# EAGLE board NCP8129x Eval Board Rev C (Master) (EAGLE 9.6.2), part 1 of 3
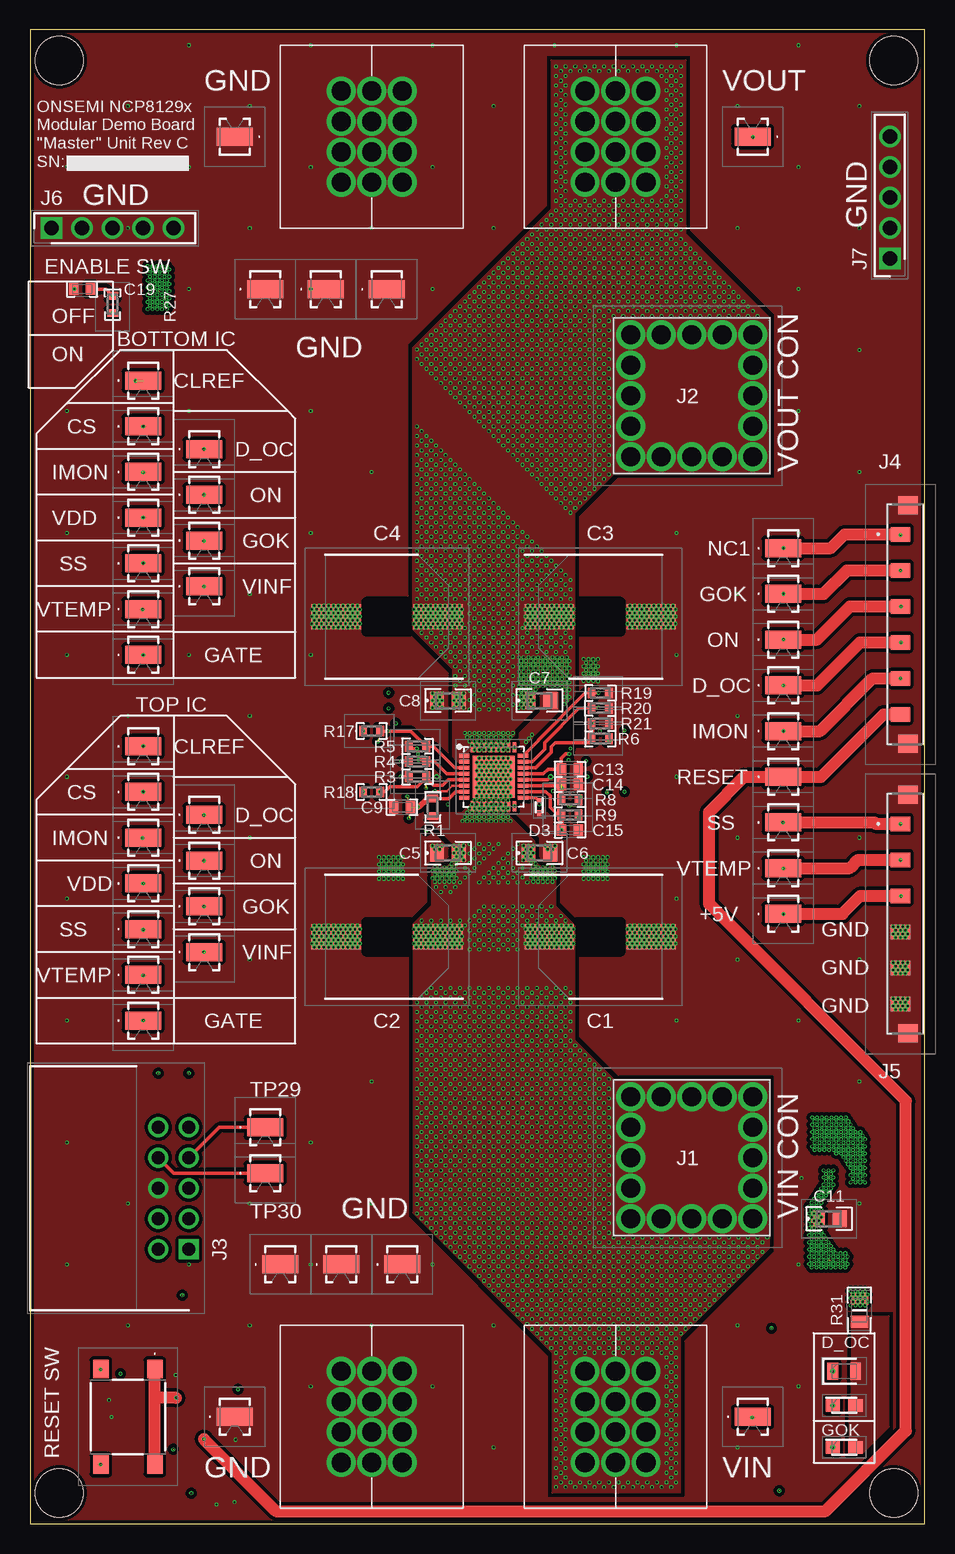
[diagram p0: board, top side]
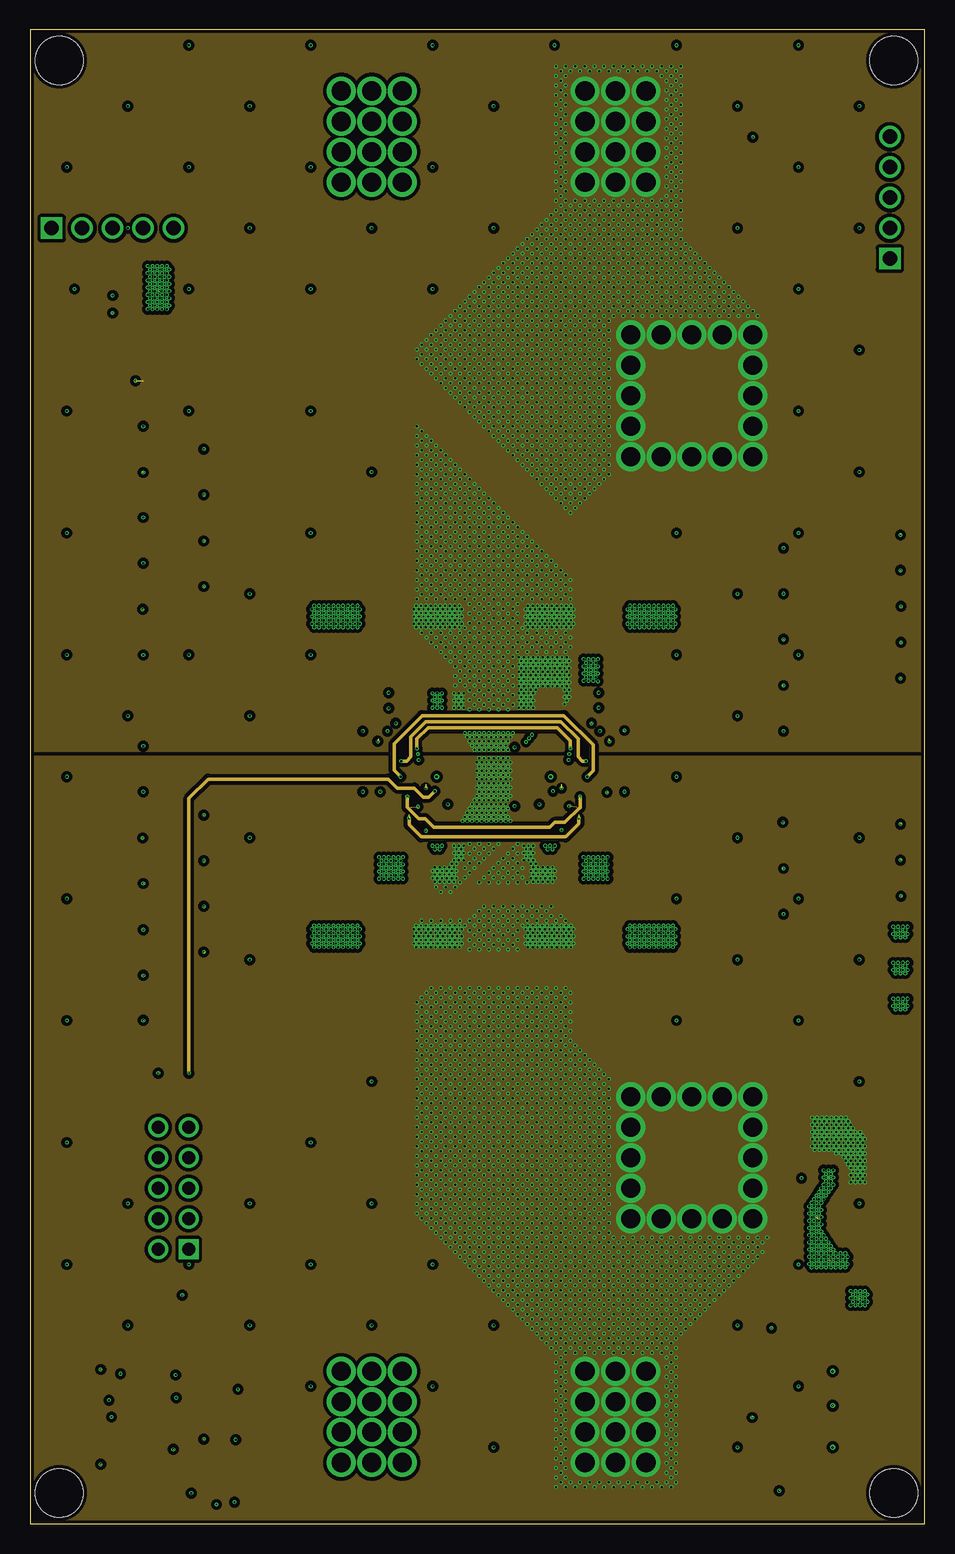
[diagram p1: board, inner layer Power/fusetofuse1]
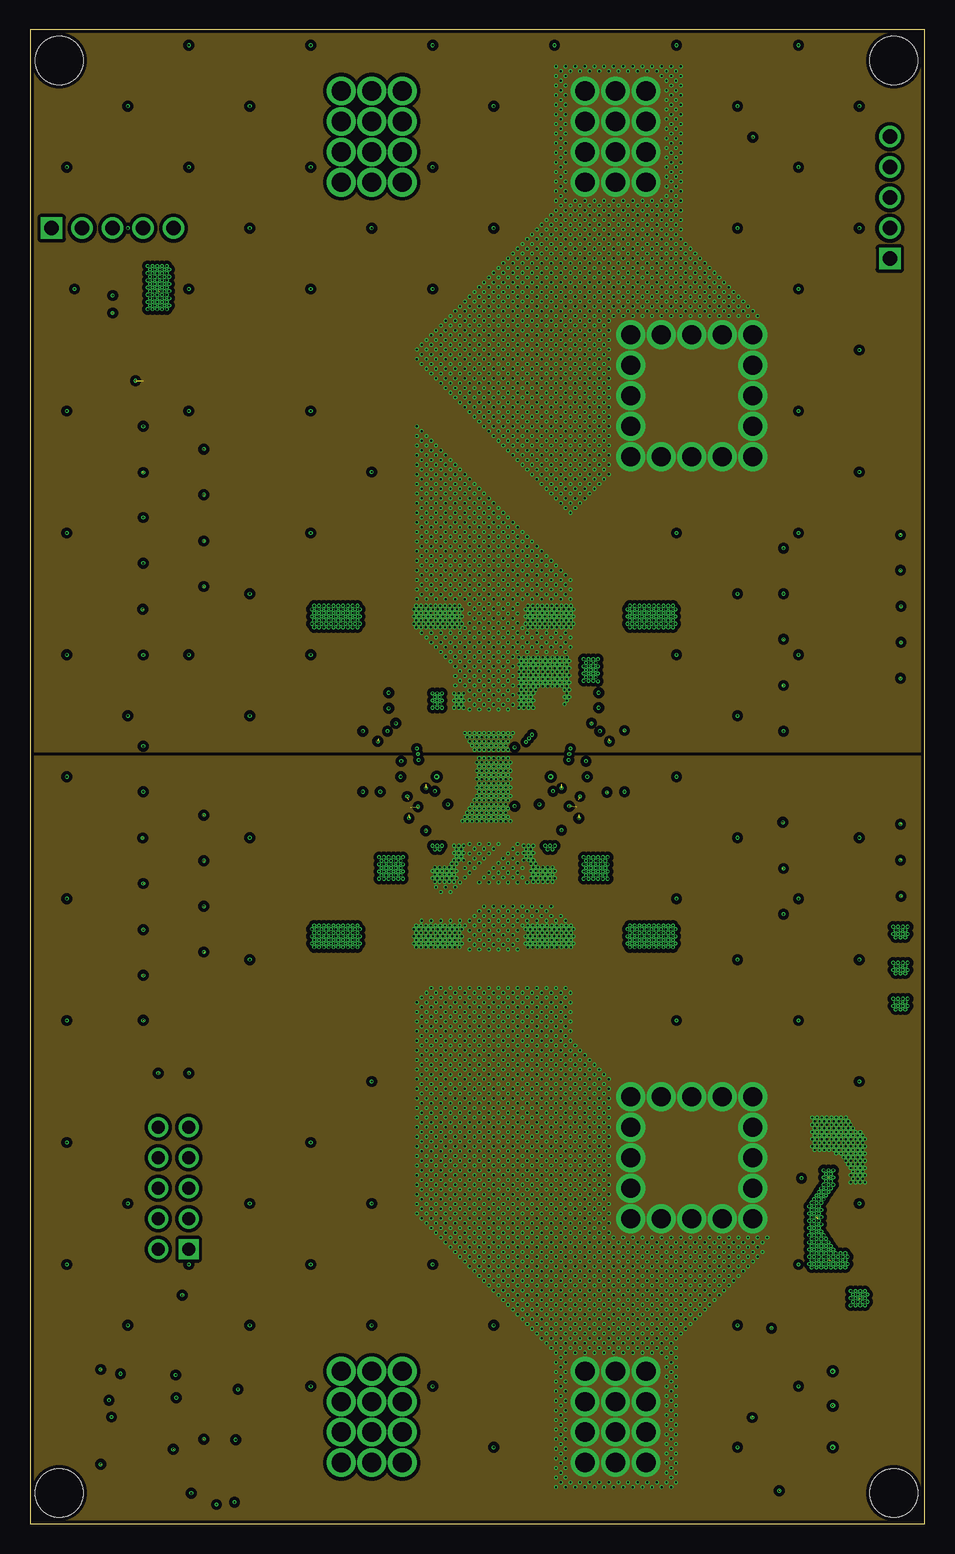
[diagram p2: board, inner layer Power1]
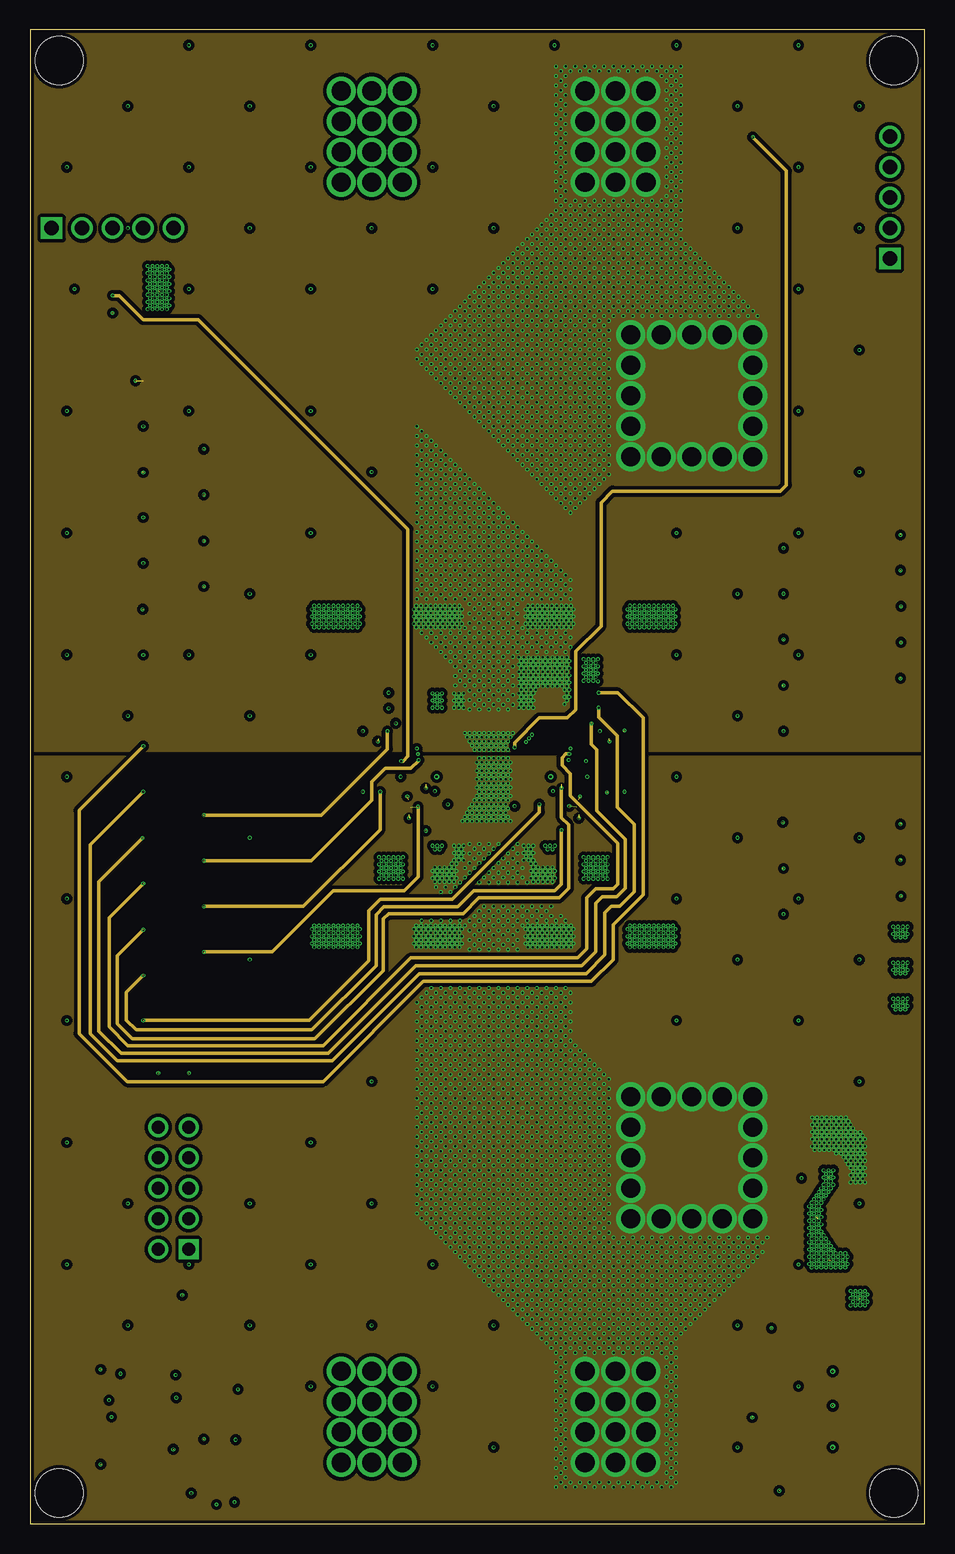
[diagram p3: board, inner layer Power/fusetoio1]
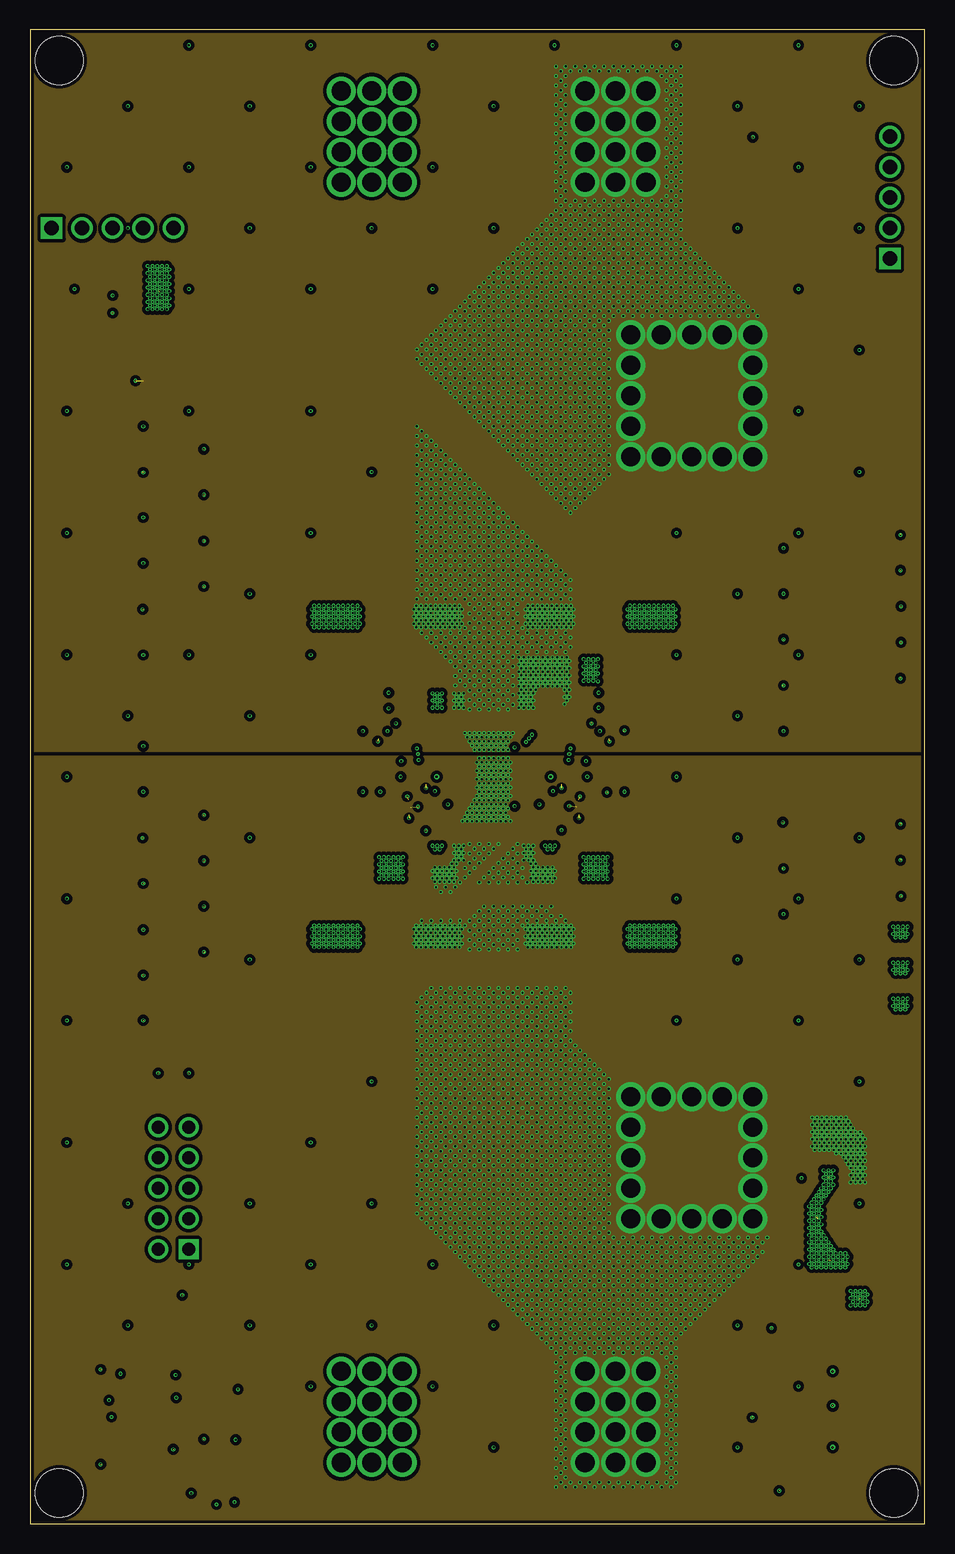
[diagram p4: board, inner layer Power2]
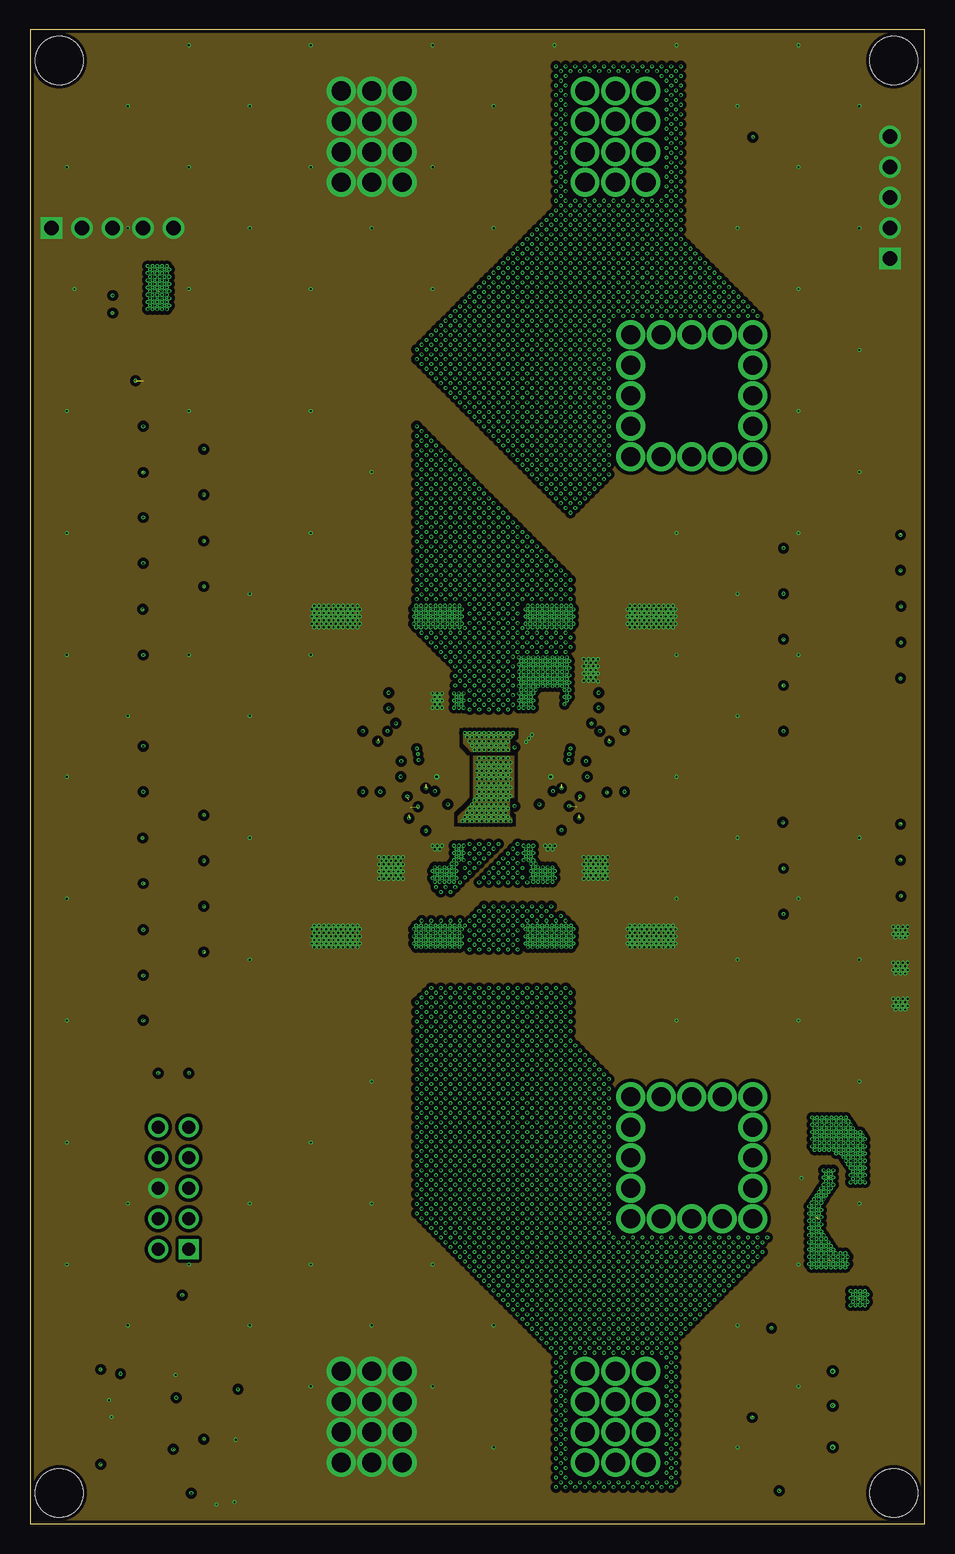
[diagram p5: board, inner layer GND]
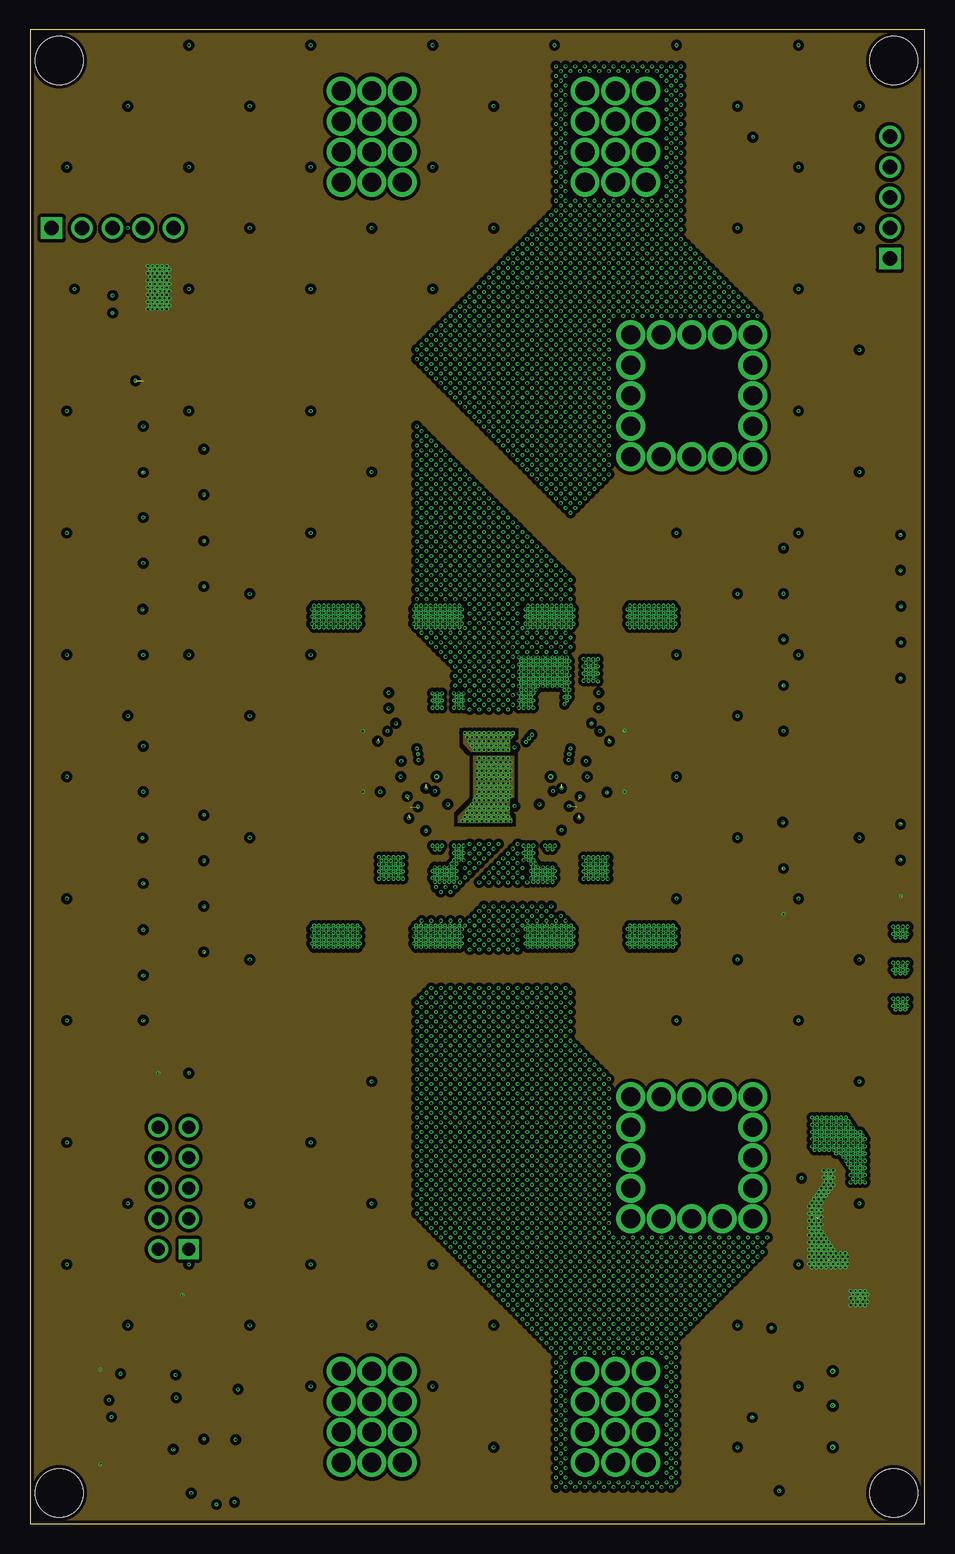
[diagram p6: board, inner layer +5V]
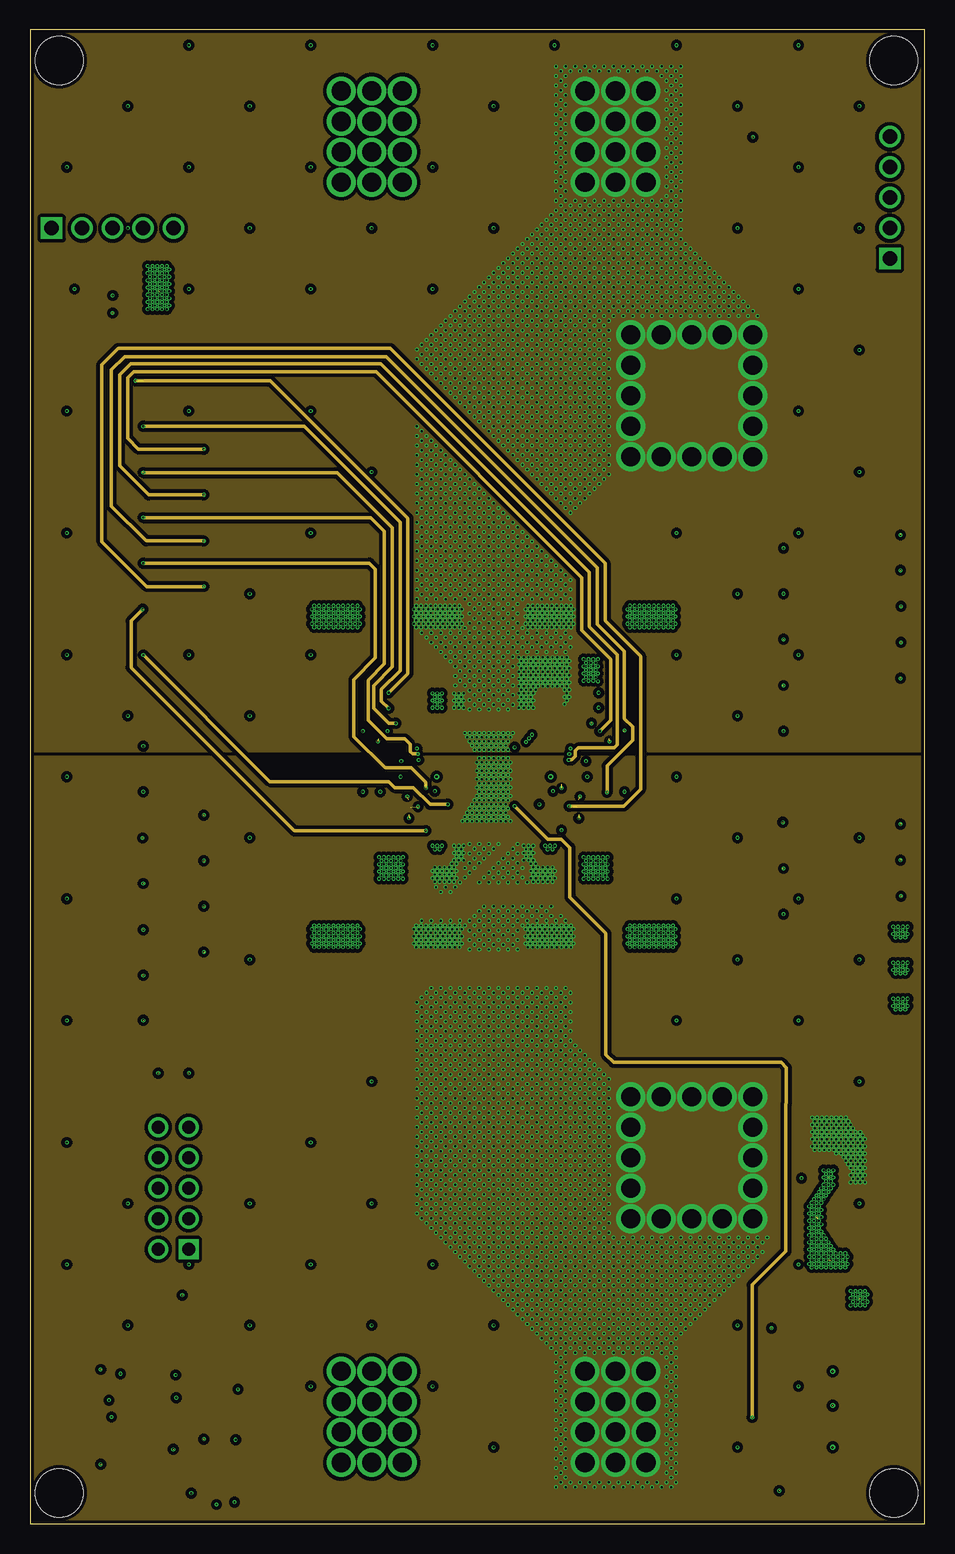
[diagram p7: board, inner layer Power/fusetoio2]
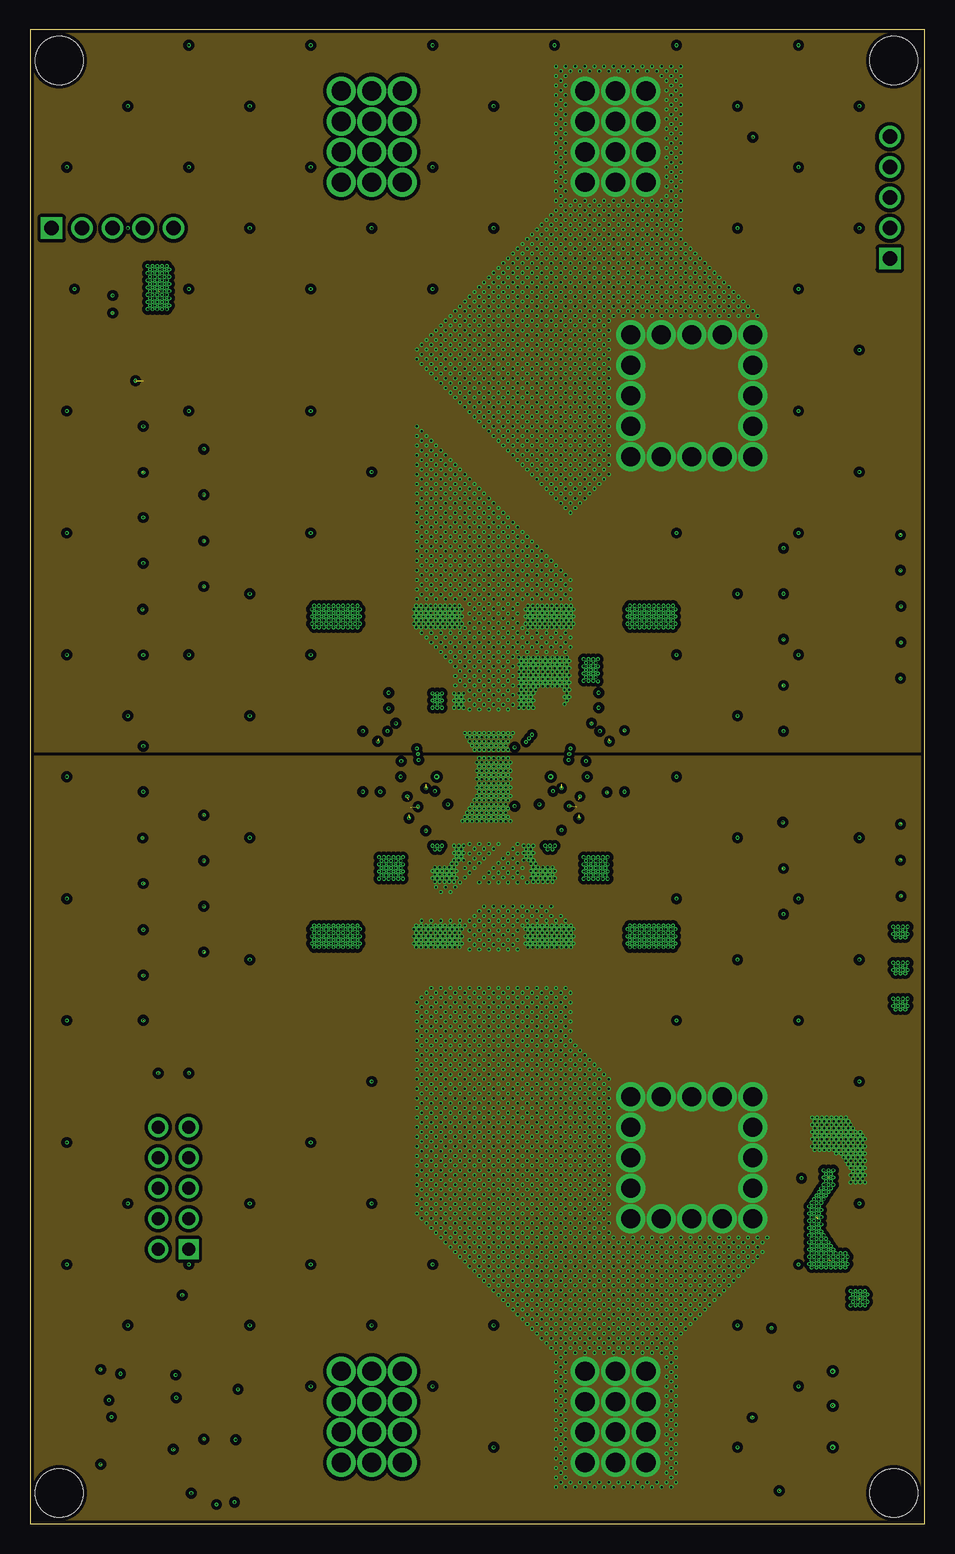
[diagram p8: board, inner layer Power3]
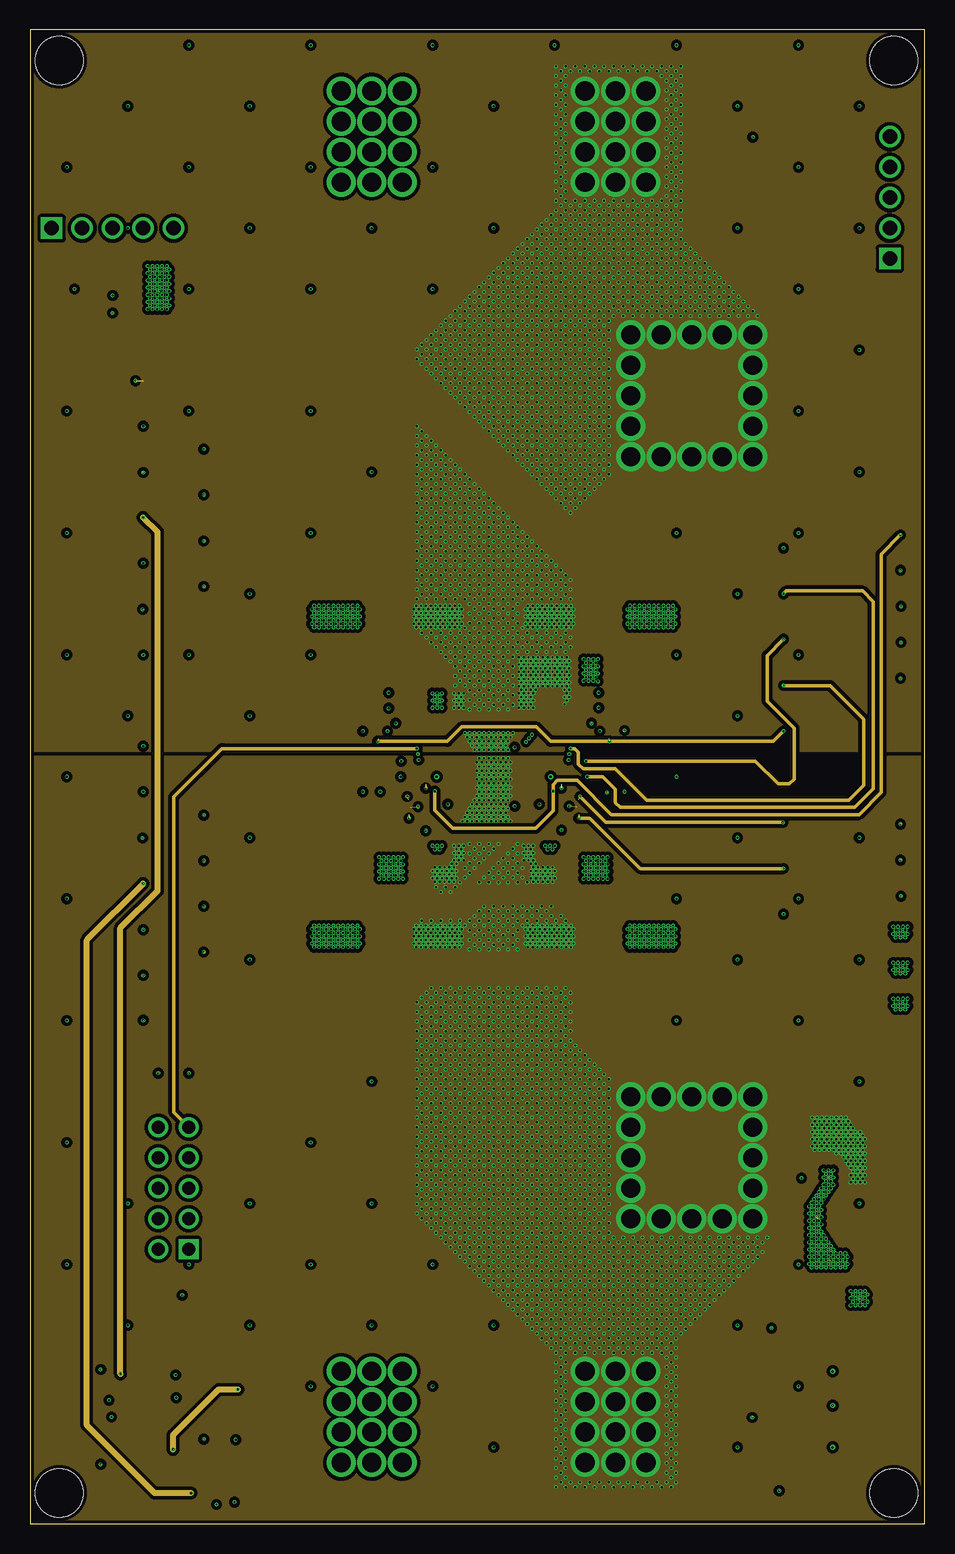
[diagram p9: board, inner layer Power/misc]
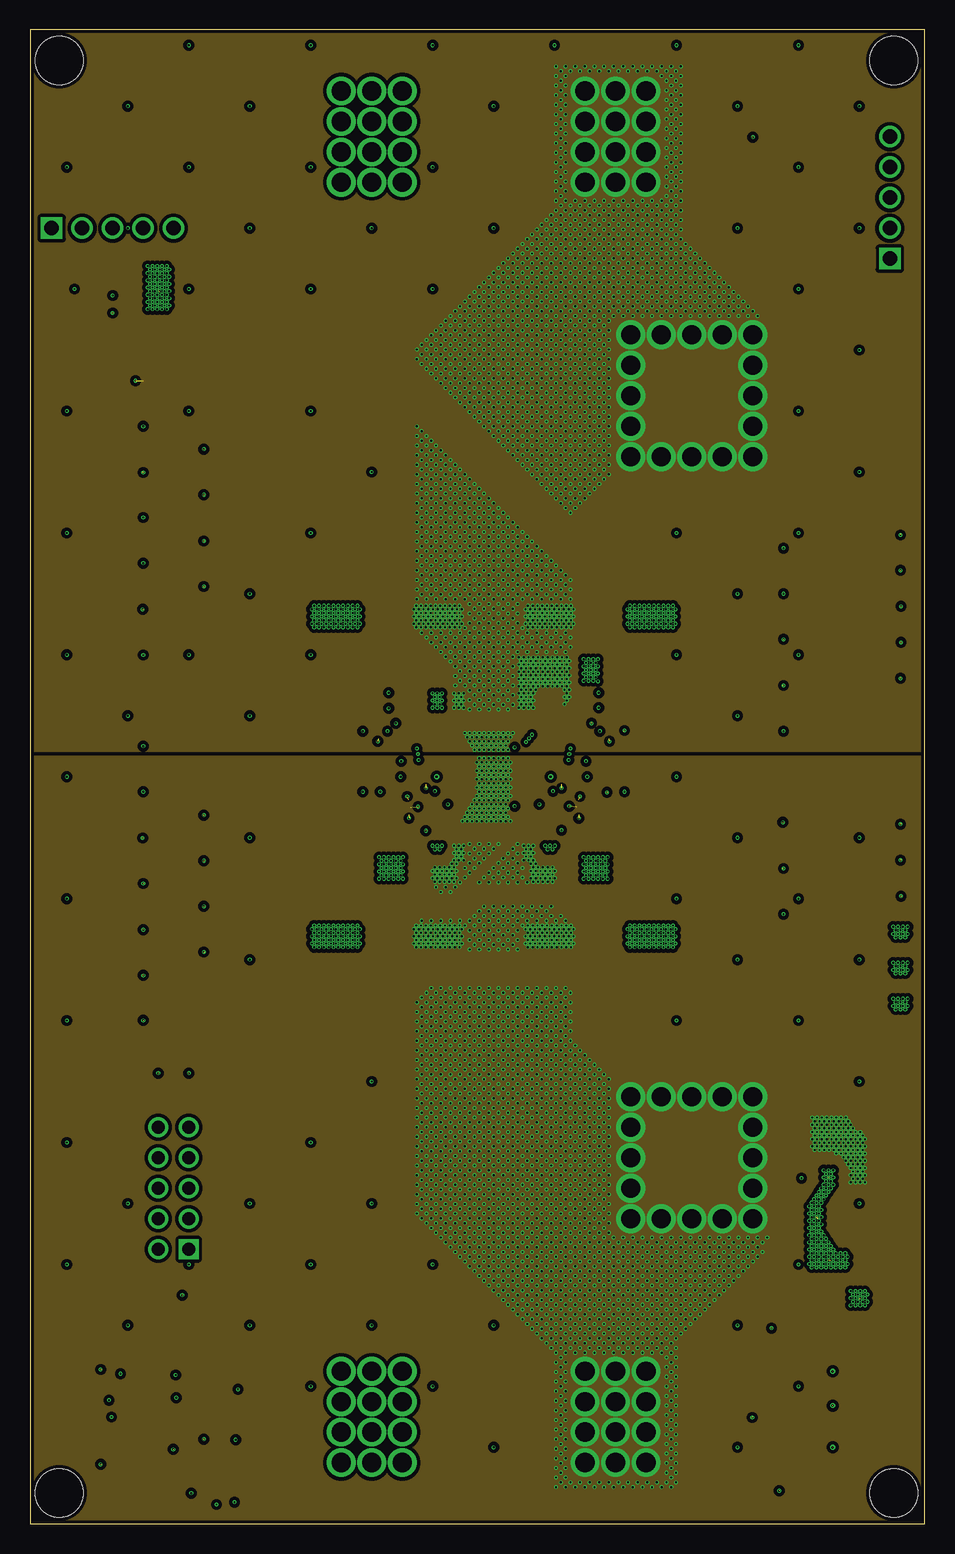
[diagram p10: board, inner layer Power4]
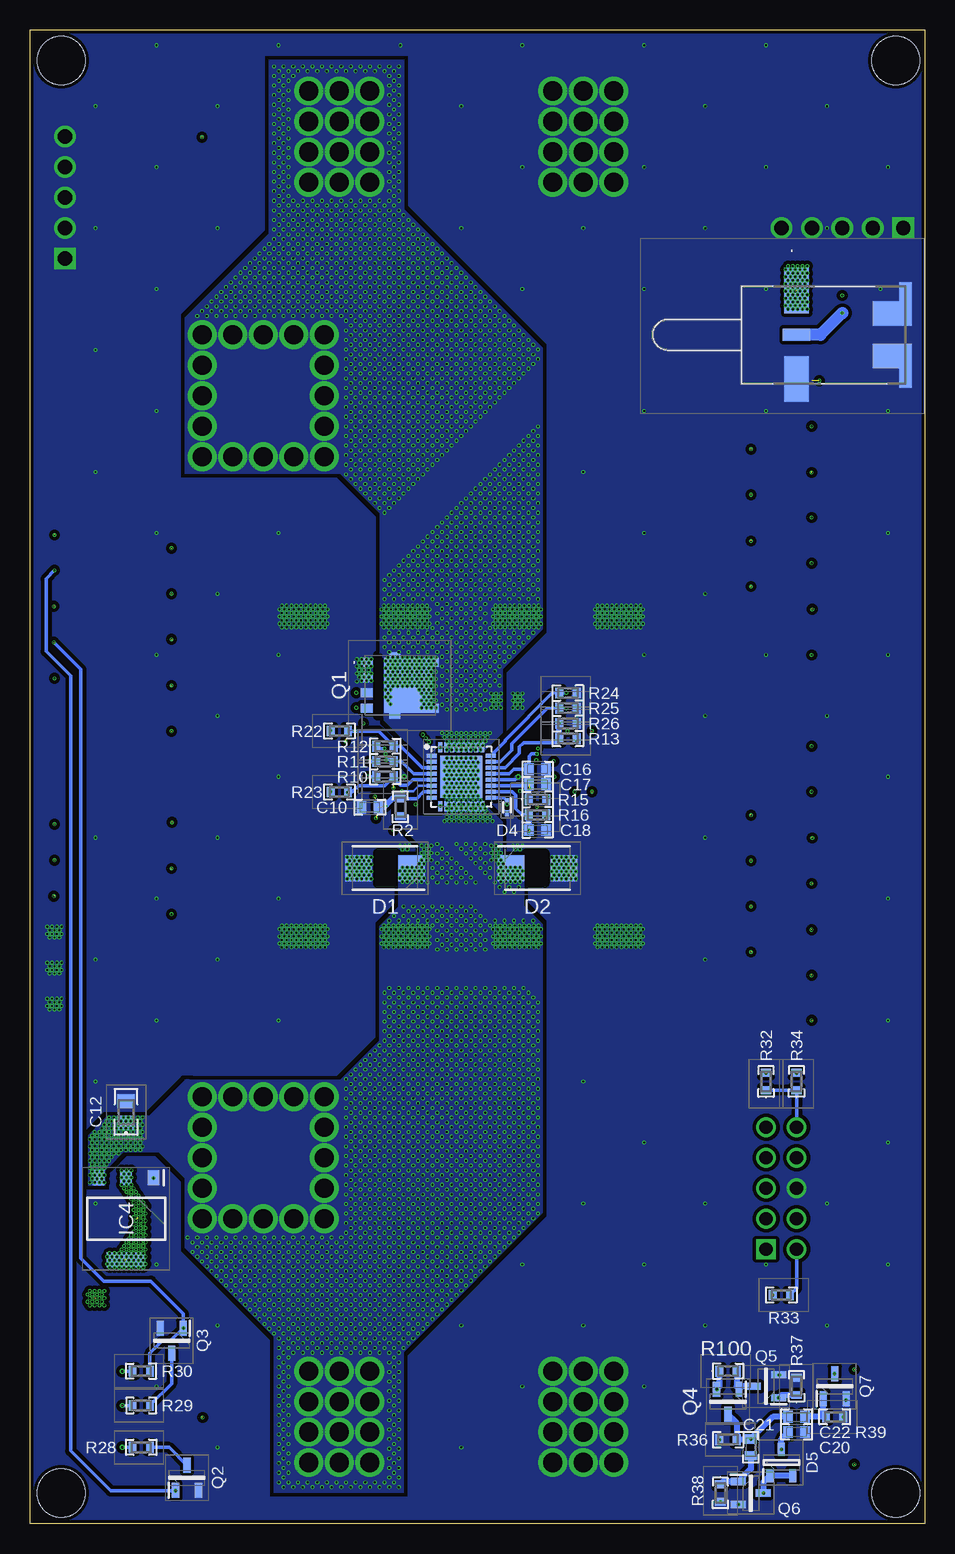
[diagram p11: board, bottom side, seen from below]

Size 74.57 x 124.46 mm. Coordinates in mm from the lower left corner, seen from the top.
Outline: 0,0 74.57,0 74.57,124.46 0,124.46 0,0
Copper layers (1+2*3+4*5+6*11+12*13+14*15+16): Top 0.035mm / dielectric 1.5mm / Power/fusetofuse1 0.035mm / dielectric 0.15mm / Power1 0.035mm / dielectric 0.2mm / Power/fusetoio1 0.035mm / dielectric 0.15mm / Power2 0.035mm / dielectric 0.2mm / GND 0.035mm / dielectric 0.15mm / +5V 0.035mm / dielectric 0.2mm / Power/fusetoio2 0.035mm / dielectric 0.15mm / Power3 0.035mm / dielectric 0.2mm / Power/misc 0.035mm / dielectric 0.15mm / Power4 0.035mm / dielectric 0.2mm / Bottom 0.035mm
Design rules "default *": minimum track width 1mil, minimum drill 0.35mm, track to track 6mil, track to pad 6mil, pad to pad 6mil, via to via 6mil, smd to smd 6mil, copper to edge 0.25mm, drill to drill 6mil, minimum pad ring 1mil, minimum via ring 1mil, stop-mask expansion 4mil, vias tented up to drill 0.3mm, thermal gap 10mil
Holes 4 mm at 2.44,121.92 71.97,121.92 2.44,2.54 71.97,2.54
tRestrict: area 28,47.6 to 31.6,50.2; area 45.6,47.6 to 49.3,50.2; area 28,74.3 to 31.6,76.8; area 45.6,74.3 to 49.3,76.8
bRestrict: area 31.6,53.3 to 33.2,55.9; area 44,53.3 to 45.6,55.9; area 45.3,67.3 to 45.6,72.4

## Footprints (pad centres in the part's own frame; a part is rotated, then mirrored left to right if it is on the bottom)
CAPAE1030X1050N = smd 4.1 x 2.05: 1 -4.25,0; 2 4.25,0
C0805 = smd 1.15 x 1.45: 1 -0.9,0; 2 0.9,0
CAPC1608X95N = smd 0.78 x 0.98: 1 -0.7,0; 2 0.7,0
DIOM5436X244N = smd 2.2 x 2.15: 1 -2.2,0; 2 2.2,0
SODFL1006X40N = smd 0.51 x 0.32: 1 -0.5,0; 2 0.5,0
SOT95P248X115-3N = smd 1.1 x 0.6: 1 -1.1,0.95; 2 -1.1,-0.95; 3 1.1,0
QFN50P500X500X140-33N = smd 0.85 x 0.3: 1 -2.45,1.75; 2 -2.45,1.25; 3 -2.45,0.75; 4 -2.45,0.25; 5 -2.45,-0.25; 6 -2.45,-0.75; 7 -2.45,-1.25; 8 -2.45,-1.75; 17 2.45,-1.75; 18 2.45,-1.25; 19 2.45,-0.75; 20 2.45,-0.25; 21 2.45,0.25; 22 2.45,0.75; 23 2.45,1.25; 24 2.45,1.75 | smd 0.3 x 0.85: 9 -1.75,-2.45; 10 -1.25,-2.45; 11 -0.75,-2.45; 12 -0.25,-2.45; 13 0.25,-2.45; 14 0.75,-2.45; 15 1.25,-2.45; 16 1.75,-2.45; 25 1.75,2.45; 26 1.25,2.45; 27 0.75,2.45; 28 0.25,2.45; 29 -0.25,2.45; 30 -0.75,2.45; 31 -1.25,2.45; 32 -1.75,2.45 | smd 3.5 x 3.5: 33 0,0
SOT230P700X180-4N = smd 1.25 x 0.95: 1 -3.4,2.3; 2 -3.4,0; 3 -3.4,-2.3 | smd 1.25 x 3.2: 4 3.4,0
7461059 = drill 1.6 pad 2.3: 1 0,0; 2 0,-2.54; 3 0,-5.08; 4 0,-7.62; 5 0,-10.16; 6 2.54,-10.16; 7 5.08,-10.16; 8 7.62,-10.16; 9 10.16,-10.16; 10 10.16,-7.62; 11 10.16,-5.08; 12 10.16,-2.54; 13 10.16,0; 14 7.62,0; 15 5.08,0; 16 2.54,0
SHDRRA10W64P254X254_2X5_2036X8 = drill 1.1 pad 1.65 square: 1 0,0 | drill 1.1 pad 1.65: 2 0,2.54; 3 2.54,0; 4 2.54,2.54; 5 5.08,0; 6 5.08,2.54; 7 7.62,0; 8 7.62,2.54; 9 10.16,0; 10 10.16,2.54
209159006101116 = smd 1.2 x 1.6: 1 -7.5,-0.38; 2 -4.5,-0.38; 3 -1.5,-0.38; 4 1.5,-0.38; 5 4.5,-0.38; 6 7.5,-0.38 | smd 1.5 x 1.6: MP1 -9.935,0.25; MP2 9.935,0.25
RHDR5W70P0X254_1X5_1310X250X86 = drill 1.2 pad 1.8 square: 1 0,0 | drill 1.2 pad 1.8: 2 2.54,0; 3 5.08,0; 4 7.62,0; 5 10.16,0
LEDM2012X80N = smd 1.2 x 1.05: 1 -0.95,0; 2 0.95,0
LEDC2012X80N = smd 0.9 x 1.4: 1 -0.95,0; 2 0.95,0
NTMFS006N12MCT1G = smd 0.75 x 1: 1 -1.905,-2.795; 2 -0.635,-2.795; 3 0.635,-2.795; 4 1.905,-2.795 | smd 4.56 x 0.425: 5 0,-1.118 | smd 5.55 x 0.905: 6 0,-0.453 | smd 4.56 x 2.725: 7 0,1.362 | smd 0.75 x 0.475: 8 1.905,2.962; 9 -1.905,2.962
SOT96P237X111-3N = smd 1.25 x 0.6: 1 -1.05,0.955; 2 -1.05,-0.955; 3 1.05,0
SOT95P237X101-3N = smd 1.25 x 0.6: 1 -1.05,0.95; 2 -1.05,-0.95; 3 1.05,0
ERJS03J155V = smd 0.65 x 0.9: 1 -0.725,0; 2 0.725,0
RESC2012X75N = smd 1 x 1.45: 1 -0.95,0; 2 0.95,0
ET01MD1SAPE = smd 3.81 x 2.03: 1 -3.685,0; 3 3.685,0 | smd 1.02 x 2.29: 2 0,0 | smd 3.63 x 1.02: MP1 -2.58,9.07; MP4 2.58,9.07 | smd 2.03 x 2.23: MP2 -1.78,7.445; MP3 1.78,7.445
430182043816 = smd 1.55 x 1.3: 1 -3.975,2.25; 2 -3.975,-2.25; 3 3.975,2.25; 4 3.975,-2.25
5191TR = smd 3 x 1.5: 1 0,0
7464000 = drill 1.6: P$1 0,2.54; P$2 0,0; P$3 0,-2.54; P$4 0,-5.08; P$5 2.54,-5.08; P$6 2.54,-2.54; P$7 2.54,0; P$8 2.54,2.54; P$9 5.08,2.54; P$10 5.08,0; P$11 5.08,-2.54; P$12 5.08,-5.08

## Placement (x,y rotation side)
C1  865230557006  [CAPAE1030X1050N]  47.52,48.89 0 top
C2  865230557006  [CAPAE1030X1050N]  29.74,48.89 180 top
C3  865230557006  [CAPAE1030X1050N]  47.52,75.56 0 top
C4  865230557006  [CAPAE1030X1050N]  29.74,75.56 180 top
C5  C0805X223K5RACTU  [C0805]  34.82,55.88 0 top
C6  C0805X223K5RACTU  [C0805]  42.44,55.88 0 top
C7  C0805X223K5RACTU  [C0805]  42.44,68.58 0 top
C8  C0805X223K5RACTU  [C0805]  34.82,68.58 0 top
C9  C0603C104K1RACAUTO  [CAPC1608X95N]  31.01,59.69 180 top
C10  C0603C104K1RACAUTO  [CAPC1608X95N]  46.25,59.69 180 bottom
C11  C0805X223K5RACTU  [C0805]  66.57,25.4 0 top
C12  C0805X223K5RACTU  [C0805]  66.57,34.29 90 bottom
C13  C0603C104K1RACAUTO  [CAPC1608X95N]  44.98,62.86 0 top
C14  C0603C104K1RACAUTO  [CAPC1608X95N]  44.98,61.59 0 top
C15  C0603C104K1RACAUTO  [CAPC1608X95N]  44.98,57.78 0 top
C16  C0603C104K1RACAUTO  [CAPC1608X95N]  32.28,62.86 0 bottom
C17  C0603C104K1RACAUTO  [CAPC1608X95N]  32.28,61.59 0 bottom
C18  C0603C104K1RACAUTO  [CAPC1608X95N]  32.28,57.78 0 bottom
C19  C0603C104K1RACAUTO  [CAPC1608X95N]  4.34,102.87 180 top
C20  C0603C104K1RACAUTO  [CAPC1608X95N]  10.69,7.62 0 bottom
C21  C0603C104K1RACAUTO  [CAPC1608X95N]  14.5,6.35 90 bottom
C22  C0603C104K1RACAUTO  [CAPC1608X95N]  10.69,8.89 180 bottom
D1  SMBJ13A  [DIOM5436X244N]  44.98,54.61 180 bottom
D2  SMBJ13A  [DIOM5436X244N]  32.28,54.61 0 bottom
D3  BAS16P2T5G  [SODFL1006X40N]  42.44,59.69 270 top
D4  BAS16P2T5G  [SODFL1006X40N]  34.82,59.69 270 bottom
D5  BAT54C-G3-08  [SOT95P248X115-3N]  11.96,5.08 90 bottom
IC1  NCP81295MNTXG  [QFN50P500X500X140-33N]  38.63,62.23 0 top
IC2  NCP81295MNTXG  [QFN50P500X500X140-33N]  38.63,62.23 0 bottom
IC4  LM1117MPX-18NOPB  [SOT230P700X180-4N]  66.57,25.4 270 bottom
J1  7461059  [7461059]  50.06,35.56 0 top
J2  7461059  [7461059]  50.06,99.06 0 top
J3  61201021721  [SHDRRA10W64P254X254_2X5_2036X8]  13.23,22.86 90 top
J4  209159006101116  [209159006101116]  72.92,74.93 270 top
J5  209159006101116  [209159006101116]  72.92,50.8 270 top
J6  M20-7820542  [RHDR5W70P0X254_1X5_1310X250X86]  1.8,107.95 0 top
J7  M20-7820542  [RHDR5W70P0X254_1X5_1310X250X86]  71.65,105.41 90 top
LED1  150080GS75000  [LEDM2012X80N]  67.84,6.35 0 top
LED2  150080GS75000  [LEDM2012X80N]  67.84,9.84 0 top
LED3  150080RS75000  [LEDC2012X80N]  67.84,12.7 0 top
Q1  NTMFS006N12MCT1G  [NTMFS006N12MCT1G]  43.71,69.85 270 bottom
Q2  2N7002LT1  [SOT96P237X111-3N]  61.49,3.81 90 bottom
Q3  2N7002LT1  [SOT96P237X111-3N]  62.76,15.24 270 bottom
Q4  NTR1P02LT1G  [SOT95P237X101-3N]  16.41,10.16 270 bottom
Q5  NTR3C21NZT1G  [SOT96P237X111-3N]  13.23,11.43 180 bottom
Q6  NTR3C21NZT1G  [SOT96P237X111-3N]  14.5,2.54 0 bottom
Q7  NTR3C21NZT1G  [SOT96P237X111-3N]  7.52,11.43 90 bottom
R1  ERJU03F56R0V  [ERJS03J155V]  33.55,59.69 270 top
R2  ERJU03F56R0V  [ERJS03J155V]  43.71,59.69 270 bottom
R3  ERJU03F56R0V  [ERJS03J155V]  32.28,62.23 0 top
R4  ERJU03F56R0V  [ERJS03J155V]  32.28,63.5 0 top
R5  ERJU03F56R0V  [ERJS03J155V]  32.28,64.77 0 top
R6  ERJU03F56R0V  [ERJS03J155V]  47.52,65.41 0 top
R8  ERJU03F56R0V  [ERJS03J155V]  44.98,60.32 0 top
R9  ERJU03F56R0V  [ERJS03J155V]  44.98,59.05 0 top
R10  ERJU03F56R0V  [ERJS03J155V]  44.98,62.23 0 bottom
R11  ERJU03F56R0V  [ERJS03J155V]  44.98,63.5 0 bottom
R12  ERJU03F56R0V  [ERJS03J155V]  44.98,64.77 0 bottom
R13  ERJU03F56R0V  [ERJS03J155V]  29.74,65.41 0 bottom
R15  ERJU03F56R0V  [ERJS03J155V]  32.28,60.32 0 bottom
R16  ERJU03F56R0V  [ERJS03J155V]  32.28,59.05 0 bottom
R17  ERJU03F56R0V  [ERJS03J155V]  28.47,66.04 0 top
R18  ERJU03F56R0V  [ERJS03J155V]  28.47,60.96 0 top
R19  ERJU03F56R0V  [ERJS03J155V]  47.52,69.22 0 top
R20  ERJU03F56R0V  [ERJS03J155V]  47.52,67.94 0 top
R21  ERJU03F56R0V  [ERJS03J155V]  47.52,66.67 0 top
R22  ERJU03F56R0V  [ERJS03J155V]  48.79,66.04 0 bottom
R23  ERJU03F56R0V  [ERJS03J155V]  48.79,60.96 0 bottom
R24  ERJU03F56R0V  [ERJS03J155V]  29.74,69.22 0 bottom
R25  ERJU03F56R0V  [ERJS03J155V]  29.74,67.94 0 bottom
R26  ERJU03F56R0V  [ERJS03J155V]  29.74,66.67 0 bottom
R27  ERJU03F56R0V  [ERJS03J155V]  6.88,101.6 90 top
R28  ERJU03F56R0V  [ERJS03J155V]  65.3,6.35 0 bottom
R29  ERJU03F56R0V  [ERJS03J155V]  65.3,9.84 0 bottom
R30  ERJU03F56R0V  [ERJS03J155V]  65.3,12.7 0 bottom
R31  ERJP6WF1303V  [RESC2012X75N]  69.11,17.78 270 top
R32  ERJU03F56R0V  [ERJS03J155V]  13.23,36.83 90 bottom
R33  ERJU03F56R0V  [ERJS03J155V]  11.96,19.05 180 bottom
R34  ERJU03F56R0V  [ERJS03J155V]  10.69,36.83 90 bottom
R36  ERJU03F56R0V  [ERJS03J155V]  16.41,6.98 180 bottom
R37  ERJU03F56R0V  [ERJS03J155V]  10.69,11.43 90 bottom
R38  ERJU03F56R0V  [ERJS03J155V]  17.04,2.54 270 bottom
R39  ERJU03F56R0V  [ERJS03J155V]  7.52,8.89 0 bottom
R100  ERJU03F56R0V  [ERJS03J155V]  16.41,12.7 0 bottom
S1  ET01MD1SAPE  [ET01MD1SAPE]  10.69,99.06 270 bottom
S2  430182043816  [430182043816]  8.15,8.89 270 top
TP1  5191TR  [5191TR]  19.58,33.02 0 top
TP2  5191TR  [5191TR]  19.58,29.21 0 top
TP3  5191TR  [5191TR]  17.04,8.89 0 top
TP4  5191TR  [5191TR]  60.22,8.89 0 top
TP5  5191TR  [5191TR]  17.04,115.57 180 top
TP6  5191TR  [5191TR]  60.22,115.57 180 top
TP7  5191TR  [5191TR]  62.76,81.28 0 top
TP8  5191TR  [5191TR]  62.76,77.47 0 top
TP9  5191TR  [5191TR]  62.76,73.66 0 top
TP10  5191TR  [5191TR]  62.76,69.85 0 top
TP11  5191TR  [5191TR]  62.76,66.04 0 top
TP12  5191TR  [5191TR]  62.76,62.23 0 top
TP13  5191TR  [5191TR]  62.76,58.42 0 top
TP14  5191TR  [5191TR]  62.76,54.61 0 top
TP15  5191TR  [5191TR]  14.5,59.05 0 top
TP16  5191TR  [5191TR]  14.5,55.24 0 top
TP17  5191TR  [5191TR]  14.5,51.43 0 top
TP18  5191TR  [5191TR]  14.5,47.62 0 top
TP19  5191TR  [5191TR]  9.42,41.91 0 top
TP20  5191TR  [5191TR]  9.42,45.72 0 top
TP21  5191TR  [5191TR]  9.42,49.53 0 top
TP22  5191TR  [5191TR]  9.42,53.34 0 top
TP23  5191TR  [5191TR]  9.42,57.15 0 top
TP24  5191TR  [5191TR]  9.42,60.96 0 top
TP25  5191TR  [5191TR]  9.42,64.77 0 top
TP26  5191TR  [5191TR]  14.5,89.53 0 top
TP27  5191TR  [5191TR]  14.5,85.72 0 top
TP28  5191TR  [5191TR]  14.5,81.91 0 top
TP29  5191TR  [5191TR]  14.5,78.1 0 top
TP30  5191TR  [5191TR]  9.42,72.39 0 top
TP31  5191TR  [5191TR]  9.42,76.2 0 top
TP32  5191TR  [5191TR]  9.42,80.01 0 top
TP33  5191TR  [5191TR]  9.42,83.82 0 top
TP34  5191TR  [5191TR]  9.42,87.63 0 top
TP35  5191TR  [5191TR]  9.42,91.44 0 top
TP36  5191TR  [5191TR]  9.42,95.25 0 top
TP37  5191TR  [5191TR]  62.76,50.8 0 top
TP38  5191TR  [5191TR]  19.58,102.87 0 top
TP39  5191TR  [5191TR]  24.66,102.87 0 top
TP40  5191TR  [5191TR]  29.74,102.87 0 top
TP41  5191TR  [5191TR]  20.85,21.59 0 top
TP42  5191TR  [5191TR]  25.93,21.59 0 top
TP43  5191TR  [5191TR]  31.01,21.59 0 top
U$1  7464000  [7464000]  25.93,10.16 0 top
U$2  7464000  [7464000]  46.25,10.16 0 top
U$3  7464000  [7464000]  25.93,116.84 0 top
U$4  7464000  [7464000]  46.25,116.84 0 top

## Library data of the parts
C1-C4 = SamacSys_Parts; DESCRIPTION: Wurth Elektronik 100uF 35 V dc Aluminium Electrolytic Capacitor, WCAP-AS5H Series 5000h 10.5 (Dia.) x 9.85mm; HEIGHT: 10.5mm; MANUFACTURER_NAME: Wurth Elektronik; MANUFACTURER_PART_NUMBER: 865230557006; MOUSER_PART_NUMBER: 710-865230557006; MOUSER_PRICE-STOCK: https://www.mouser.co.uk/ProductDetail/Wurth-Elektronik/865230557006?qs=0KOYDY2FL28VdE9DUGoPjQ%3D%3D
C5-C8 C11 C12 = SamacSys_Parts; ARROW_PART_NUMBER: C0805X223K5RACTU; ARROW_PRICE-STOCK: https://www.arrow.com/en/products/c0805x223k5ractu/kemet-corporation?region=nac; DESCRIPTION: SMD Comm X7R Flex, Ceramic, 0.022 uF, 10%, 50 VDC, 125 VDC, 125?C, -55?C, X7R, SMD, MLCC, FT-CAP, Temperature Stable, 2.5 % , 45.4545 GOhms, 13 mg, 0805, 2mm, 1.25mm, 0.78mm, 0.75mm, 0.5mm, 4000, 78 Weeks, 80; HEIGHT: 1.1mm; MANUFACTURER_NAME: KEMET; MANUFACTURER_PART_NUMBER: C0805X223K5RACTU; MOUSER_PART_NUMBER: 80-C0805X223K5R; MOUSER_PRICE-STOCK: https://www.mouser.co.uk/ProductDetail/KEMET/C0805X223K5RACTU?qs=p6yRp5s%252B%2FXRyuzEkovIpgw%3D%3D
C9 C10 C13-C22 = SamacSys_Parts; DESCRIPTION: SMD Auto X7R, Ceramic, 0.1 uF, 10%, 100 VDC, X7R, SMD, MLCC, Temperature Stable, Automotive Grade, 0603; HEIGHT: 0.95mm; MANUFACTURER_NAME: KEMET; MANUFACTURER_PART_NUMBER: C0603C104K1RACAUTO; MOUSER_PART_NUMBER: 80-C0603C104K1RAUTO; MOUSER_PRICE-STOCK: https://www.mouser.co.uk/ProductDetail/KEMET/C0603C104K1RACAUTO?qs=3Rah4i%252BhyCGTQ5uPNXtfZA%3D%3D
D1 D2 = SamacSys_Parts; DESCRIPTION: Diode TVS Single Uni-Dir 13V 600W 2-Pin SMB T/R; HEIGHT: 2.44mm; MANUFACTURER_NAME: LITTELFUSE; MANUFACTURER_PART_NUMBER: SMBJ13A; MOUSER_PART_NUMBER: 576-SMBJ13A; MOUSER_PRICE-STOCK: https://www.mouser.co.uk/ProductDetail/Littelfuse/SMBJ13A?qs=HR2RnyOI4E7jYyaNBU0w0w%3D%3D
D3 D4 = SamacSys_Parts; DESCRIPTION: Diodes - General Purpose, Power, Switching SWITCHING DIODE SOD923; HEIGHT: 0.4mm; MANUFACTURER_NAME: onsemi; MANUFACTURER_PART_NUMBER: BAS16P2T5G; MOUSER_PART_NUMBER: 863-BAS16P2T5G; MOUSER_PRICE-STOCK: https://www.mouser.co.uk/ProductDetail/onsemi/BAS16P2T5G?qs=xGcJQ%252BnsJwsOIzUKPy5pxg%3D%3D
D5 = SamacSys_Parts; DESCRIPTION: Vishay BAT54C-G3-08, Dual SMT Schottky Small Signal Diode, Common Cathode, 30V 200mA, 5ns, 3-Pin SOT-23; HEIGHT: 1.15mm; MANUFACTURER_NAME: Vishay; MANUFACTURER_PART_NUMBER: BAT54C-G3-08; MOUSER_PART_NUMBER: 78-BAT54C-G3-08; MOUSER_PRICE-STOCK: https://www.mouser.co.uk/ProductDetail/Vishay-Semiconductors/BAT54C-G3-08?qs=KP8Io%2FXyE5QQ%2FZAl3kVl1Q%3D%3D
IC1 IC2 = SamacSys_Parts; ARROW_PART_NUMBER: NCP81295MNTXG; ARROW_PRICE-STOCK: https://www.arrow.com/en/products/ncp81295mntxg/on-semiconductor; DESCRIPTION: HOT SWAP SMART FUSE; HEIGHT: 1.4mm; MANUFACTURER_NAME: onsemi; MANUFACTURER_PART_NUMBER: NCP81295MNTXG; MOUSER_PART_NUMBER: 863-NCP81295MNTXG; MOUSER_PRICE-STOCK: https://www.mouser.co.uk/ProductDetail/onsemi/NCP81295MNTXG?qs=W0yvOO0ixfEM9uhw2julAQ%3D%3D
IC4 = SamacSys_Parts; DESCRIPTION: Available in 1.8 V, 2.5 V, 3.3 V, 5 V, and Adjustable Versions; Space-saving SOT-223 package; Current limiting and thermal protection; Output current: 800 mA; Line regulation: 0.2% (maximum); Load regulation: 0.4% (maximum); HEIGHT: 1.8mm; MANUFACTURER_NAME: onsemi; MANUFACTURER_PART_NUMBER: LM1117MPX-18NOPB; MOUSER_PART_NUMBER: 863-LM1117MPX-18NOPB; MOUSER_PRICE-STOCK: https://www.mouser.co.uk/ProductDetail/onsemi/LM1117MPX-18NOPB?qs=DPoM0jnrROWLfPqSDvF0mA%3D%3D
J1 J2 = SamacSys_Parts; DESCRIPTION: Wurth Elektronik, Brass Screw Terminal, 240A; HEIGHT: 13.5mm; MANUFACTURER_NAME: Wurth Elektronik; MANUFACTURER_PART_NUMBER: 7461059; MOUSER_PART_NUMBER: 710-7461059; MOUSER_PRICE-STOCK: https://www.mouser.co.uk/ProductDetail/Wurth-Elektronik/7461059?qs=wr8lucFkNMXpCcsX18jYrg%3D%3D
J3 = SamacSys_Parts; DESCRIPTION: 10way 2.54mm male box Header right angle Wurth Elektronik WR-BHD Series, 2.54mm Pitch 10 Way 2 Row Shrouded Right Angle PCB Header, Surface Mount; HEIGHT: 9.1mm; MANUFACTURER_NAME: Wurth Elektronik; MANUFACTURER_PART_NUMBER: 61201021721; MOUSER_PART_NUMBER: 710-61201021721; MOUSER_PRICE-STOCK: https://www.mouser.co.uk/ProductDetail/Wurth-Elektronik/61201021721?qs=ZtY9WdtwX5567gkupD2iFg%3D%3D
J4 J5 = SamacSys_Parts; DESCRIPTION: Board to Board & Mezzanine Connectors Horizontal Sockt6Way 3mm Pitch 5A 125VAC; HEIGHT: 3mm; MANUFACTURER_NAME: Kyocera AVX; MANUFACTURER_PART_NUMBER: 209159006101116; MOUSER_PART_NUMBER: 581-209159006101116; MOUSER_PRICE-STOCK: https://www.mouser.co.uk/ProductDetail/KYOCERA-AVX/209159006101116?qs=b4vKS93X7SwcdpXWffJnjQ%3D%3D
J6 J7 = SamacSys_Parts; DESCRIPTION: Headers & Wire Housings 5 PIN SIL VERTICAL SOCKET GOLD+TIN; HEIGHT: 8.65mm; MANUFACTURER_NAME: Harwin; MANUFACTURER_PART_NUMBER: M20-7820542; MOUSER_PART_NUMBER: 855-M20-7820542; MOUSER_PRICE-STOCK: https://www.mouser.co.uk/ProductDetail/Harwin/M20-7820542?qs=vF78I%252BjhbY9JoekBTXVWnQ%3D%3D
LED1 LED2 = SamacSys_Parts; DESCRIPTION: 150080GS75000, Wurth Elektronik WL-SMCW 520 nm Green LED, 2012 (0805) Clear SMD package; HEIGHT: 0.8mm; MANUFACTURER_NAME: Wurth Elektronik; MANUFACTURER_PART_NUMBER: 150080GS75000; MOUSER_PART_NUMBER: 710-150080GS75000; MOUSER_PRICE-STOCK: https://www.mouser.co.uk/ProductDetail/Wurth-Elektronik/150080GS75000?qs=2kOmHSv6VfQRoTEZVk1mGA%3D%3D
LED3 = SamacSys_Parts; DESCRIPTION: LED,Wurth Elektronik,150080RS75000 Wurth Elektronik 150080RS75000, WL-SMCW Series Red LED, 625 nm 2012 (0805) Clear, Rectangle Lens SMD package; HEIGHT: 0.8mm; MANUFACTURER_NAME: Wurth Elektronik; MANUFACTURER_PART_NUMBER: 150080RS75000; MOUSER_PART_NUMBER: 710-150080RS75000; MOUSER_PRICE-STOCK: https://www.mouser.co.uk/ProductDetail/Wurth-Elektronik/150080RS75000?qs=LlUlMxKIyB2jdCo7bnfgew%3D%3D
Q1 = SamacSys_Parts; DESCRIPTION: ON Semiconductor NTMFS006N12MCT1G; HEIGHT: 1.1mm; MANUFACTURER_NAME: onsemi; MANUFACTURER_PART_NUMBER: NTMFS006N12MCT1G; MOUSER_PART_NUMBER: 863-NTMFS006N12MCT1G; MOUSER_PRICE-STOCK: https://www.mouser.co.uk/ProductDetail/onsemi/NTMFS006N12MCT1G?qs=HBWAp0VN4Ri6NIfu80r37A%3D%3D
Q2 Q3 = SamacSys_Parts; DESCRIPTION: MOSFET N-CH 60V 115MA SOT23-3; HEIGHT: 1.11mm; MANUFACTURER_NAME: onsemi; MANUFACTURER_PART_NUMBER: 2N7002LT1; MOUSER_PART_NUMBER: 863-2N7002LT1; MOUSER_PRICE-STOCK: https://www.mouser.co.uk/ProductDetail/onsemi/2N7002LT1?qs=vLkC5FC1VN%2FcwI%252Bf34Z4TQ%3D%3D
Q4 = SamacSys_Parts; DESCRIPTION: Small Signal MOSFET -20V -1.3A 220 mOhm Single P-Channel SOT-23 Logic Level; HEIGHT: 1.01mm; MANUFACTURER_NAME: onsemi; MANUFACTURER_PART_NUMBER: NTR1P02LT1G; MOUSER_PART_NUMBER: 863-NTR1P02LT1G; MOUSER_PRICE-STOCK: https://www.mouser.co.uk/ProductDetail/onsemi/NTR1P02LT1G?qs=ZXBb0xZ9WeCGH3oHt9wcQg%3D%3D
Q5-Q7 = SamacSys_Parts; DESCRIPTION: ON SEMICONDUCTOR - NTR3C21NZT1G - MOSFET, N-CH, 20V, 3.6A, SOT-23; HEIGHT: 1.11mm; MANUFACTURER_NAME: onsemi; MANUFACTURER_PART_NUMBER: NTR3C21NZT1G; MOUSER_PART_NUMBER: 863-NTR3C21NZT1G; MOUSER_PRICE-STOCK: https://www.mouser.co.uk/ProductDetail/onsemi/NTR3C21NZT1G?qs=tCMd4XlZ%2FiDqlfJKftdpPA%3D%3D
R1-R6 R8-R13 R15-R30 R32-R34 R36-R39 R100 = SamacSys_Parts; DESCRIPTION: Panasonic ERJU03 Series Thick Film Resistor 0603 Case 56 0.1W +/-100ppm/C; HEIGHT: 0.55mm; MANUFACTURER_NAME: Panasonic; MANUFACTURER_PART_NUMBER: ERJU03F56R0V
R31 = SamacSys_Parts; ARROW_PART_NUMBER: ERJP6WF1303V; ARROW_PRICE-STOCK: https://www.arrow.com/en/products/erj-p6wf1303v/panasonic; DESCRIPTION: Panasonic ERJP6W Series Thick Film Surface Mount Fixed Resistor 0805 Case 130k +/-1% 0.5W +/-200ppm/C; HEIGHT: 0.75mm; MANUFACTURER_NAME: Panasonic; MANUFACTURER_PART_NUMBER: ERJP6WF1303V
S1 = SamacSys_Parts; DESCRIPTION: Toggle Switches ON None ON SPDT 20VAC 20VDC 0.4W; HEIGHT: 5.72mm; MANUFACTURER_NAME: C & K COMPONENTS; MANUFACTURER_PART_NUMBER: ET01MD1SAPE; MOUSER_PART_NUMBER: 611-ET01MD1SAPE; MOUSER_PRICE-STOCK: https://www.mouser.co.uk/ProductDetail/CK/ET01MD1SAPE?qs=pYvtfcBFDEzTOYrckHtWUQ%3D%3D
S2 = SamacSys_Parts; DESCRIPTION: Black Tactile Switch, Single Pole Single Throw (SPST) 50 mA @ 12 V dc 0.9mm Surface Mount; HEIGHT: 4.45mm; MANUFACTURER_NAME: Wurth Elektronik; MANUFACTURER_PART_NUMBER: 430182043816; MOUSER_PART_NUMBER: 710-430182043816; MOUSER_PRICE-STOCK: https://www.mouser.co.uk/ProductDetail/Wurth-Elektronik/430182043816?qs=wr8lucFkNMVm%252BwK7rSM84A%3D%3D
TP1-TP43 = SamacSys_Parts; DESCRIPTION: Circuit Board Hardware - PCB TEST POINT (BLACK) ON TAPE AND REEL; HEIGHT: 2.63mm; MANUFACTURER_NAME: Keystone Electronics; MANUFACTURER_PART_NUMBER: 5191TR; MOUSER_PART_NUMBER: 534-5191TR; MOUSER_PRICE-STOCK: https://www.mouser.co.uk/ProductDetail/Keystone-Electronics/5191TR?qs=vLWxofP3U2z5ZV%2FXGVtphA%3D%3D
U$1-U$4 = SamacSys_Parts

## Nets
+5V: C11.1 IC4.2 IC4.4 J5.3 R17.1 R18.1 R22.1 R23.1 R31.1 R33.2 R34.2 S1.1 S2.2 S2.4 TP37.1
+5V_LED: LED1.2 LED2.2 LED3.2 R31.2
CLREF1: IC1.24 R19.1 TP25.1
CLREF2: IC2.24 R24.1 TP36.1
CS1: IC1.23 R20.1 TP24.1
CS2: IC2.23 R25.1 TP35.1
D_OC: J3.9 J4.4 Q3.1 R5.1 R12.1 R30.2 TP10.1
D_OC1: IC1.3 R5.2 R17.2 TP15.1
D_OC2: IC2.3 R12.2 R22.2 TP26.1
GATE1: D3.1 IC1.17 TP19.1
GATE2: D4.1 IC2.17 TP30.1
GND: C1.2 C2.2 C3.2 C4.2 C5.1 C6.2 C7.2 C8.1 C9.2 C10.2 C11.2 C12.2 C13.2 C14.2 C15.2 C16.2 C17.2 C18.2 C19.2 C20.2 D1.2 D2.2 D3.2 D4.2 IC1.20 IC2.20 IC4.1 J3.6 J4.MP1 J4.MP2 J5.4 J5.5 J5.6 J5.MP1 J5.MP2 J6.1 J6.2 J6.3 J6.4 J6.5 J7.1 J7.2 J7.3 J7.4 J7.5 Q1.1 Q1.2 Q1.3 Q2.2 Q3.2 Q5.2 Q6.2 Q7.2 R19.2 R20.2 R21.2 R24.2 R25.2 R26.2 R36.2 R37.2 R38.2 R39.2 S1.3 S1.MP1 S1.MP2 S1.MP3 S1.MP4 TP3.1 TP5.1 TP38.1 TP39.1 TP40.1 TP41.1 TP42.1 TP43.1 U$1.P$1 U$1.P$2 U$1.P$3 U$1.P$4 U$1.P$5 U$1.P$6 U$1.P$7 U$1.P$8 U$1.P$9 U$1.P$10 U$1.P$11 U$1.P$12 U$3.P$1 U$3.P$2 U$3.P$3 U$3.P$4 U$3.P$5 U$3.P$6 U$3.P$7 U$3.P$8 U$3.P$9 U$3.P$10 U$3.P$11 U$3.P$12
GOK: J4.2 Q2.1 R3.1 R10.1 TP8.1
GOK1: IC1.5 R3.2 R18.2 TP17.1
GOK2: IC2.5 R10.2 R23.2 TP28.1
IMON: J4.5 R6.2 R13.2 TP11.1
IMON1: IC1.22 R6.1 R21.1 TP23.1
IMON2: IC2.22 R13.1 R26.1 TP34.1
MASTER_RESET: Q5.1 R37.1 S2.1 S2.3
N$1: LED1.1 R28.1
N$2: Q2.3 R28.2
N$3: Q3.3 R29.2
N$4: LED2.1 R29.1
N$5: LED3.1 R30.1
N$6: J3.10 R32.1 R34.1
N$7: J3.2 R33.1
N$8: C20.1 D5.3 Q4.2 R100.1
N$9: Q4.1 Q5.3 R100.2
N$11: C21.1 Q6.1 R38.1
N$12: C22.1 Q7.1 R39.1
ON: C19.1 J4.3 R4.1 R11.1 R27.2 TP9.1
ON1: IC1.4 R4.2 TP16.1
ON2: IC2.4 R11.2 TP27.1
ON_PRE_RES: R27.1 S1.2
SDA: IC1.6 IC2.6 J4.1 R32.2 TP7.1
SLAVE_RESET: C21.2 C22.2 J4.6 Q4.3 R36.1 TP12.1
SS: J5.1 R8.2 R15.2 TP13.1
SS1: C14.1 IC1.19 R8.1 TP21.1
SS2: C17.1 IC2.19 R15.1 TP32.1
TP29: J3.7 TP1.1
TP30: J3.8 TP2.1
VDD1: C13.1 D5.1 D5.2 IC1.21 Q6.3 TP22.1
VDD2: C16.1 IC2.21 Q7.3 TP33.1
VIN: C1.1 C2.1 C5.2 C6.1 C12.1 D1.1 D2.1 IC1.9 IC1.10 IC1.11 IC1.12 IC1.13 IC1.14 IC1.15 IC1.33 IC2.10 IC2.11 IC2.12 IC2.13 IC2.14 IC2.15 IC2.16 IC2.33 IC4.3 J1.1 J1.2 J1.3 J1.4 J1.5 J1.6 J1.7 J1.8 J1.9 J1.10 J1.11 J1.12 J1.13 J1.14 J1.15 J1.16 R1.2 R2.2 U$2.P$1 U$2.P$2 U$2.P$3 U$2.P$4 U$2.P$5 U$2.P$6 U$2.P$7 U$2.P$8 U$2.P$9 U$2.P$10 U$2.P$11 U$2.P$12
VIN_S: IC1.16 IC2.9 TP4.1
VINF1: C9.1 IC1.7 R1.1 TP18.1
VINF2: C10.1 IC2.7 R2.1 TP29.1
VOUT: C3.1 C4.1 C7.1 C8.2 IC1.1 IC1.2 IC1.26 IC1.27 IC1.28 IC1.29 IC1.30 IC1.31 IC1.32 IC2.1 IC2.2 IC2.25 IC2.26 IC2.27 IC2.28 IC2.29 IC2.30 IC2.31 J2.1 J2.2 J2.3 J2.4 J2.5 J2.6 J2.7 J2.8 J2.9 J2.10 J2.11 J2.12 J2.13 J2.14 J2.15 J2.16 Q1.5 Q1.6 Q1.7 Q1.8 Q1.9 U$4.P$1 U$4.P$2 U$4.P$3 U$4.P$4 U$4.P$5 U$4.P$6 U$4.P$7 U$4.P$8 U$4.P$9 U$4.P$10 U$4.P$11 U$4.P$12
VOUT_S: IC1.25 IC2.32 TP6.1
VTEMP: J5.2 R9.2 R16.2 TP14.1
VTEMP1: C15.1 IC1.18 R9.1 TP20.1
VTEMP2: C18.1 IC2.18 R16.1 TP31.1

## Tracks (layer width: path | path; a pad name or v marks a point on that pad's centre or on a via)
+5V  (via drill 0.15 pad 0.3)  (14 unrouted)
  Top 1: TP37.1 67.7,50.8 69.2,52.3 J5.3
  other vias: 27.73,66.03 27.73,60.98 49.53,66.08 49.53,60.98 65.13,23.73 65.53,23.73 65.93,23.73 65.73,23.43 65.33,23.43 64.93,23.43 65.13,23.13 65.53,23.13 65.93,23.13 65.73,22.83 65.33,22.83 64.93,22.83 65.33,24.03 65.73,24.03 64.93,24.03 65.93,24.33 65.53,24.33 65.13,24.33 65.33,24.63 65.73,24.63 64.93,24.63 65.53,24.93 65.93,24.93 65.13,24.93 65.33,25.23 64.93,25.23 65.73,25.23 65.93,25.53 65.53,25.53 65.13,25.53 64.93,25.83 65.33,25.83 65.73,25.83 65.93,26.13 65.53,26.13 65.13,26.13 68.58,19.08 68.98,19.08 69.38,19.08 69.78,19.08 68.78,18.78 69.18,18.78 69.58,18.78 68.38,18.78 68.58,18.48 68.98,18.48 69.38,18.48 69.78,18.48 68.78,18.18 69.18,18.18 69.58,18.18 68.38,18.18 68.78,19.38 68.38,19.38 69.18,19.38 69.58,19.38 62.78,50.78 72.58,52.28 9.8,104.8 10.2,104.8 10.6,104.8 11,104.8 11.4,104.8 10,104.5 10.4,104.5 10.8,104.5 11.2,104.5 11.6,104.5 9.8,104.2 10.2,104.2 10.6,104.2 11,104.2 11.4,104.2 10,103.9 10.4,103.9 10.8,103.9 11.2,103.9 11.6,103.9 11.4,103.6 11,103.6 10.6,103.6 10.2,103.6 9.8,103.6 10,103.3 10.4,103.3 10.8,103.3 11.2,103.3 11.6,103.3 9.8,103 10.2,103 10.6,103 11,103 11.4,103 10,102.7 10.4,102.7 10.8,102.7 11.2,102.7 11.6,102.7 9.8,102.4 10.2,102.4 10.6,102.4 11,102.4 11.4,102.4 10,102.1 10.4,102.1 10.8,102.1 11.2,102.1 11.6,102.1 9.8,101.8 10.2,101.8 10.6,101.8 11,101.8 11.4,101.8 10,101.5 10.4,101.5 10.8,101.5 11.2,101.5 11.6,101.5 9.8,101.2 10.2,101.2 10.6,101.2 11,101.2 11.4,101.2 12.68,19.03 10.68,37.53 5.88,12.83 5.88,4.93 65.13,22.53 65.53,22.53 64.93,22.23 65.33,22.23 65.73,22.23 65.13,21.93 65.53,21.93 64.93,21.63 65.33,21.63 65.73,21.63 65.13,21.33 65.53,21.33 65.93,21.93 65.93,22.53 66.13,22.23 66.13,22.83 66.33,22.53 66.13,24.03 66.13,23.43 66.33,23.13 65.93,21.33 66.13,21.63 66.33,21.93 66.33,21.33 66.53,21.63 66.53,22.23 66.73,21.93 66.73,22.53 66.73,21.33 67.13,21.33 67.53,21.33 67.93,21.33 68.13,21.63 67.73,21.63 67.33,21.63 66.93,21.63 67.13,21.93 67.53,21.93 67.93,21.93 66.93,22.23 67.33,22.23 67.73,22.23 68.13,22.23 67.13,22.53 67.53,22.53 67.93,22.53 66.53,22.83 66.33,23.73 66.53,23.43 66.73,23.13 66.93,22.83 65.33,26.43 65.73,26.43 65.53,26.73 65.13,26.73 64.93,26.43 65.93,26.73 65.73,27.03 65.33,27.03 66.13,27.03 65.53,27.33 65.93,27.33 66.33,27.33 65.73,27.63 66.13,27.63 66.53,27.63 66.33,27.93 65.93,27.93 66.73,27.93 66.53,28.23 66.13,28.23 66.93,28.23 66.33,28.53 66.73,28.53 66.53,28.83 66.93,28.83 66.13,28.83 66.33,29.13 66.73,29.13 66.53,29.43 66.93,29.43 66.13,29.43
  pour +5V (isolate 0.3, rank 2, no thermals): -0.74,124.46 -0.74,0 75.46,0 75.46,124.46
+5V_LED
  pour Top (no thermals): 68.43,17.28 68.43,13.53 68.38,13.48 68.38,9.58 68.23,9.43 68.23,5.85 69.38,5.85 71.58,8.05 71.58,17.28
CLREF1  (via drill 0.15 pad 0.3)  (1 unrouted)
  Top 0.3: IC1.24 42.33,65.23 42.33,65.28 46.27,69.22 R19.1 47.37,69.22 v47.38,69.23
  Power/fusetoio1 0.3: v9.43,64.78 4.08,59.43 4.08,40.83 8.08,36.83 24.43,36.83 32.78,45.18 46.78,45.18 48.58,46.98 48.58,49.88 51.08,52.38 51.08,67.13 48.98,69.23 v47.38,69.23
CLREF2  (via drill 0.15 pad 0.3)  (1 unrouted)
  Power/fusetoio2 0.3: v8.8,95.23 20.03,95.23 31.48,83.78 31.48,70.83 v29.88,69.23
  Bottom 0.3: IC2.24 34.98,65.18 34.98,65.28 31.05,69.22 R24.1 29.9,69.22 v29.88,69.23
CS1  (via drill 0.15 pad 0.3)  (1 unrouted)
  Top 0.3: IC1.23 41.83,63.48 42.88,64.53 42.88,65.08 45.75,67.94 R20.1 46.83,67.98 v47.38,67.98
  Power/fusetoio1 0.3: v9.43,60.98 5.03,56.58 5.03,40.83 7.28,38.58 25.18,38.58 32.43,45.83 46.33,45.83 47.88,47.38 47.88,50.88 48.43,51.43 49.13,51.43 50.33,52.63 50.33,58.28 48.93,59.68 48.93,65.63 47.38,67.18 v47.38,67.98
CS2  (via drill 0.15 pad 0.3)  (1 unrouted)
  Power/fusetoio2 0.3: v9.43,91.43 22.83,91.43 30.83,83.43 30.83,71.08 29.28,69.53 29.28,68.53 v29.88,67.93
  Bottom 0.3: IC2.23 35.38,63.48 34.43,64.43 34.43,64.98 31.47,67.94 R25.1 v29.88,67.93
D_OC  (via drill 0.15 pad 0.3)  (3 unrouted)
  Top 0.3: v32.23,64.58 31.75,64.58 R5.1
  Top 1: TP10.1 65.6,69.85 69.18,73.43 J4.4
  Power/fusetofuse1 0.3: v32.23,64.58 32.23,65.38 33.18,66.33 43.93,66.33 45.03,65.23 v45.03,64.58
  Power/misc 0.3: v45.03,64.58 45.38,64.58 45.68,64.28 45.68,63.28 46.08,62.88 48.78,62.88 51.38,60.28 68.23,60.28 69.48,61.53 69.48,67.03 66.68,69.83 v62.78,69.83 | J3.9 11.98,34.27 11.98,60.58 15.98,64.58 v32.23,64.58
  Bottom 0.3: R30.2 64.58,14.18 63.53,15.23 62.87,15.23 Q3.1 | R12.1 45.52,64.58 v45.03,64.58 | v72.58,73.43 70.33,71.18 70.33,22.11 68.42,20.2 64.5,20.2 61.78,17.48 v61.78,16.28
D_OC1  (via drill 0.15 pad 0.3)  (1 unrouted)
  Top 0.3: IC1.3 35.38,62.98 33.59,64.77 R5.2 31.74,66.04 v29.79,66.04 v29.78,66.03 29.21,66.03 R17.2
  Power/fusetoio1 0.3: v14.48,59.03 24.28,59.03 29.78,64.53 v29.78,66.03
D_OC2  (via drill 0.15 pad 0.3)  (1 unrouted)
  Power/fusetoio2 0.3: v14.48,89.53 9.03,89.53 8.13,90.43 8.13,95.48 8.63,95.98 28.83,95.98 45.98,78.83 45.98,74.43 48.38,72.03 48.38,66.93 v47.48,66.03
  Bottom 0.3: IC2.3 41.88,62.98 43.67,64.77 R12.2 45.53,66.04 v47.47,66.04 v47.48,66.03 48.06,66.03 R22.2
GATE1  (via drill 0.15 pad 0.3)  (1 unrouted)
  Top 0.3: IC1.17 42.15,60.48 D3.1 v42.44,59.93
  Power/fusetoio1 0.3: v9.43,41.93 23.28,41.93 28.23,46.88 28.23,51.08 29.18,52.03 35.19,52.03 42.44,59.28 v42.44,59.93
GATE2  (via drill 0.15 pad 0.3)  (1 unrouted)
  Power/fusetoio2 0.3: v9.43,72.38 19.98,61.83 29.88,61.83 30.38,61.33 31.93,61.33 33.33,59.93 v34.82,59.93
  Bottom 0.3: IC2.17 35.11,60.48 D4.1 v34.82,59.93
GND  (via drill 0.15 pad 0.3, 0.2 pad 0.4)
  Top 0.3: IC1.20 43.13,61.98 v43.38,62.23
  Bottom 0.3: IC2.20 34.13,61.98 v33.88,62.23
  other vias: 27.28,76.48 26.88,76.48 26.48,76.48 26.08,76.48 25.68,76.48 25.28,76.48 24.88,76.48 24.48,76.48 24.08,76.48 23.68,76.48 27.08,76.18 26.68,76.18 26.28,76.18 25.88,76.18 25.48,76.18 25.08,76.18 24.68,76.18 23.88,76.18 24.28,76.18 23.48,76.18 27.48,76.18 23.68,75.88 24.08,75.88 24.48,75.88 24.88,75.88 25.28,75.88 25.68,75.88 26.08,75.88 26.48,75.88 26.88,75.88 27.28,75.88 23.48,75.58 23.88,75.58 24.28,75.58 24.68,75.58 25.08,75.58 25.48,75.58 25.88,75.58 26.28,75.58 26.68,75.58 27.08,75.58 27.48,75.58 23.68,75.28 24.08,75.28 24.48,75.28 24.88,75.28 25.28,75.28 25.68,75.28 26.08,75.28 26.48,75.28 26.88,75.28 27.28,75.28 23.48,74.98 23.88,74.98 24.28,74.98 24.68,74.98 25.08,74.98 25.48,74.98 25.88,74.98 26.28,74.98 26.68,74.98 27.08,74.98 27.48,74.98 27.28,74.68 26.88,74.68 26.48,74.68 26.08,74.68 25.68,74.68 23.68,74.68 24.08,74.68 24.48,74.68 24.88,74.68 25.28,74.68 53.58,76.48 53.18,76.48 52.78,76.48 52.38,76.48 51.98,76.48 51.58,76.48 51.18,76.48 50.78,76.48 50.38,76.48 49.98,76.48 53.38,76.18 52.98,76.18 52.58,76.18 52.18,76.18 51.78,76.18 51.38,76.18 50.98,76.18 50.18,76.18 50.58,76.18 49.78,76.18 53.78,76.18 49.98,75.88 50.38,75.88 50.78,75.88 51.18,75.88 51.58,75.88 51.98,75.88 52.38,75.88 52.78,75.88 53.18,75.88 53.58,75.88 49.78,75.58 50.18,75.58 50.58,75.58 50.98,75.58 51.38,75.58 51.78,75.58 52.18,75.58 52.58,75.58 52.98,75.58 53.38,75.58 53.78,75.58 49.98,75.28 50.38,75.28 50.78,75.28 51.18,75.28 51.58,75.28 51.98,75.28 52.38,75.28 52.78,75.28 53.18,75.28 53.58,75.28 49.78,74.98 50.18,74.98 50.58,74.98 50.98,74.98 51.38,74.98 51.78,74.98 52.18,74.98 52.58,74.98 52.98,74.98 53.38,74.98 53.78,74.98 53.58,74.68 53.18,74.68 52.78,74.68 52.38,74.68 51.98,74.68 49.98,74.68 50.38,74.68 50.78,74.68 51.18,74.68 51.58,74.68 53.58,49.83 53.18,49.83 52.78,49.83 52.38,49.83 51.98,49.83 51.58,49.83 51.18,49.83 50.78,49.83 50.38,49.83 49.98,49.83 53.38,49.53 52.98,49.53 52.58,49.53 52.18,49.53 51.78,49.53 51.38,49.53 50.98,49.53 50.18,49.53 50.58,49.53 49.78,49.53 53.78,49.53 49.98,49.23 50.38,49.23 50.78,49.23 51.18,49.23 51.58,49.23 51.98,49.23 52.38,49.23 52.78,49.23 53.18,49.23 53.58,49.23 49.78,48.93 50.18,48.93 50.58,48.93 50.98,48.93 51.38,48.93 51.78,48.93 52.18,48.93 52.58,48.93 52.98,48.93 53.38,48.93 53.78,48.93 49.98,48.63 50.38,48.63 50.78,48.63 51.18,48.63 51.58,48.63 51.98,48.63 52.38,48.63 52.78,48.63 53.18,48.63 53.58,48.63 49.78,48.33 50.18,48.33 50.58,48.33 50.98,48.33 51.38,48.33 51.78,48.33 52.18,48.33 52.58,48.33 52.98,48.33 53.38,48.33 53.78,48.33 53.58,48.03 53.18,48.03 52.78,48.03 52.38,48.03 51.98,48.03 49.98,48.03 50.38,48.03 50.78,48.03 51.18,48.03 51.58,48.03 27.28,49.83 26.88,49.83 26.48,49.83 26.08,49.83 25.68,49.83 25.28,49.83 24.88,49.83 24.48,49.83 24.08,49.83 23.68,49.83 27.08,49.53 26.68,49.53 26.28,49.53 25.88,49.53 25.48,49.53 25.08,49.53 24.68,49.53 23.88,49.53 24.28,49.53 23.48,49.53 27.48,49.53 23.68,49.23 24.08,49.23 24.48,49.23 24.88,49.23 25.28,49.23 25.68,49.23 26.08,49.23 26.48,49.23 26.88,49.23 27.28,49.23 23.48,48.93 23.88,48.93 24.28,48.93 24.68,48.93 25.08,48.93 25.48,48.93 25.88,48.93 26.28,48.93 26.68,48.93 27.08,48.93 27.48,48.93 23.68,48.63 24.08,48.63 24.48,48.63 24.88,48.63 25.28,48.63 25.68,48.63 26.08,48.63 26.48,48.63 26.88,48.63 27.28,48.63 23.48,48.33 23.88,48.33 24.28,48.33 24.68,48.33 25.08,48.33 25.48,48.33 25.88,48.33 26.28,48.33 26.68,48.33 27.08,48.33 27.48,48.33 27.28,48.03 26.88,48.03 26.48,48.03 26.08,48.03 25.68,48.03 23.68,48.03 24.08,48.03 24.48,48.03 24.88,48.03 25.28,48.03 34.33,69.18 33.93,69.18 33.53,69.18 33.73,68.88 34.13,68.88 33.53,68.58 33.93,68.58 34.33,68.58 33.73,68.28 34.13,68.28 33.53,67.98 33.93,67.98 34.33,67.98 34.33,56.48 33.93,56.48 33.53,56.48 33.73,56.18 34.13,56.18 42.93,56.48 43.33,56.48 43.73,56.48 43.53,56.18 43.13,56.18 31.08,55.53 30.68,55.53 30.28,55.53 29.88,55.53 29.48,55.53 29.08,55.53 30.88,55.23 30.48,55.23 30.08,55.23 29.68,55.23 29.28,55.23 29.08,54.93 29.48,54.93 29.88,54.93 30.28,54.93 30.68,54.93 31.08,54.93 29.28,54.63 29.68,54.63 30.08,54.63 30.48,54.63 30.88,54.63 29.08,54.33 29.48,54.33 29.88,54.33 30.28,54.33 30.68,54.33 31.08,54.33 29.28,54.03 29.68,54.03 30.08,54.03 30.48,54.03 30.88,54.03 29.08,53.73 29.48,53.73 29.88,53.73 30.28,53.73 30.68,53.73 31.08,53.73 48.13,55.53 47.73,55.53 47.33,55.53 46.93,55.53 46.53,55.53 46.13,55.53 47.93,55.23 47.53,55.23 47.13,55.23 46.73,55.23 46.33,55.23 46.13,54.93 46.53,54.93 46.93,54.93 47.33,54.93 47.73,54.93 48.13,54.93 46.33,54.63 46.73,54.63 47.13,54.63 47.53,54.63 47.93,54.63 46.13,54.33 46.53,54.33 46.93,54.33 47.33,54.33 47.73,54.33 48.13,54.33 46.33,54.03 46.73,54.03 47.13,54.03 47.53,54.03 47.93,54.03 46.13,53.73 46.53,53.73 46.93,53.73 47.33,53.73 47.73,53.73 48.13,53.73 46.13,72.03 46.53,72.03 46.93,72.03 47.33,72.03 46.33,71.73 46.73,71.73 47.13,71.73 46.13,71.43 46.53,71.43 46.93,71.43 47.33,71.43 46.33,71.13 46.73,71.13 47.13,71.13 46.13,70.83 46.53,70.83 46.93,70.83 47.33,70.83 46.33,70.53 46.73,70.53 47.13,70.53 46.13,70.23 46.53,70.23 46.93,70.23 47.33,70.18 13.23,123.19 23.39,123.19 33.55,123.19 43.71,123.19 53.87,123.19 64.03,123.19 8.15,118.11 18.31,118.11 38.63,118.11 58.95,118.11 69.11,118.11 64.03,113.03 33.55,113.03 23.39,113.03 13.23,113.03 3.07,113.03 8.15,107.95 18.31,107.95 28.47,107.95 38.63,107.95 58.95,107.95 69.11,107.95 64.03,102.87 33.55,102.87 23.39,102.87 13.23,102.87 3.71,102.87 69.11,97.79 64.03,92.71 23.39,92.71 13.23,92.71 3.07,92.71 69.11,87.63 28.47,87.63 64.03,82.55 53.87,82.55 23.39,82.55 3.07,82.55 58.95,77.47 18.31,77.47 3.07,72.39 13.23,72.39 23.39,72.39 53.87,72.39 64.03,72.39 8.15,67.31 18.31,67.31 58.95,67.31 3.07,62.23 53.87,62.23 18.31,57.15 58.95,57.15 69.11,57.15 3.07,52.07 53.87,52.07 64.03,52.07 18.31,46.99 58.95,46.99 69.11,46.99 3.07,41.91 53.87,41.91 64.03,41.91 28.47,36.83 69.11,36.83 3.07,31.75 23.39,31.75 8.15,26.67 18.31,26.67 28.47,26.67 69.11,26.67 3.07,21.59 13.23,21.59 23.39,21.59 33.55,21.59 64.03,21.59 8.15,16.51 18.31,16.51 28.47,16.51 38.63,16.51 58.95,16.51 23.39,11.43 33.55,11.43 64.03,11.43 38.63,6.35 58.95,6.35 71.93,49.73 72.33,49.73 72.73,49.73 73.13,49.73 72.13,49.43 72.53,49.43 72.93,49.43 71.93,49.13 72.33,49.13 72.73,49.13 73.13,49.13 72.13,48.83 72.53,48.83 72.93,48.83 71.93,46.73 72.33,46.73 72.73,46.73 73.13,46.73 72.13,46.43 72.53,46.43 72.93,46.43 71.93,46.13 72.33,46.13 72.73,46.13 73.13,46.13 72.13,45.83 72.53,45.83 72.93,45.83 71.93,43.73 72.33,43.73 72.73,43.73 73.13,43.73 72.13,43.43 72.53,43.43 72.93,43.43 71.93,43.13 72.33,43.13 72.73,43.13 73.13,43.13 72.13,42.83 72.53,42.83 72.93,42.83 15.53,1.58 17.03,1.78 6.58,10.28 6.78,8.88 12.13,12.38 17.13,6.98 41.33,65.13 41.58,65.43 41.83,65.73 64.28,28.78
  pour GND (isolate 0.3, rank 2, no thermals): -0.74,124.46 -0.74,0 75.46,0 75.46,124.46
  pour Top (isolate 0.3, rank 2, no thermals): -0.74,124.46 -0.74,0 75.46,0 75.46,124.46
  pour Bottom (isolate 0.3, rank 2, no thermals): -0.74,124.46 -0.74,0 75.46,0 75.46,124.46
GOK  (via drill 0.15 pad 0.3)  (3 unrouted)
  Top 0.3: R3.1 v30.88,62.23
  Top 1: TP8.1 66.12,77.47 68.08,79.43 J4.2
  Power/fusetofuse1 0.3: v30.88,62.23 30.33,62.78 30.33,64.98 32.68,67.33 44.48,67.33 46.93,64.88 46.93,62.73 v46.43,62.23
  Power/misc 0.3: v46.43,62.23 47.73,62.23 48.78,61.18 48.78,60.08 49.18,59.68 68.73,59.68 70.28,61.23 70.28,76.83 69.38,77.73 63.03,77.73 v62.78,77.48
  Bottom 0.3: R10.1 v46.43,62.23 | v62.43,2.73 67.86,2.73 71.18,6.05 71.18,70.63 73.23,72.68 73.23,78.73 v72.53,79.43
GOK1  (via drill 0.15 pad 0.3)  (2 unrouted)
  Top 0.3: R18.2 29.56,60.96 29.98,61.38 32.28,61.38 33.01,62.1 R3.2 33.01,62.13 33.61,61.53 34.38,61.53 34.83,61.98 IC1.5
  Power/fusetoio1 0.3: v14.48,51.43 22.78,51.43 29.18,57.83 v29.18,60.98
GOK2  (via drill 0.15 pad 0.3)  (2 unrouted)
  Power/fusetoio2 0.3: v14.48,81.88 9.68,81.88 6.78,84.78 6.78,96.13 7.88,97.23 29.68,97.23 47.28,79.63 47.28,74.93 49.53,72.68 49.53,67.08 50.23,66.38 50.23,65.28 48.08,63.13 v48.08,60.93
  Bottom 0.3: R23.2 47.7,60.96 47.19,61.48 45.01,61.48 R10.2 44.26,62.05 43.73,61.53 43.13,61.53 42.68,61.98 IC2.5
IMON  (via drill 0.15 pad 0.3)  (4 unrouted)
  Top 1: TP11.1 65.84,66.04 70.23,70.43 J4.5
  Power/misc 0.3: v28.98,65.18 34.78,65.18 35.98,66.38 42.18,66.38 43.38,65.18 v48.28,65.18 61.93,65.18 v62.78,66.03
  other vias: 72.53,70.43
IMON1  (via drill 0.15 pad 0.3)  (2 unrouted)
  Top 0.3: IC1.22 42.13,62.98 43.43,64.28 43.43,64.73 43.76,65.05 46.45,65.05 R6.1
  Top 0.5: R6.1 R21.1
  Power/fusetoio1 0.3: v9.38,57.13 5.73,53.48 5.73,41.03 7.58,39.18 24.83,39.18 32.13,46.48 45.98,46.48 47.13,47.63 47.13,51.68 47.68,52.23 48.88,52.23 49.58,52.93 49.58,57.03 47.23,59.38 47.23,64.48 46.78,64.93 v46.78,66.68
IMON2  (via drill 0.15 pad 0.3)  (2 unrouted)
  Power/fusetoio2 0.3: v9.43,87.58 25.58,87.58 30.18,82.98 30.18,71.38 28.63,69.83 28.63,67.93 29.88,66.68 v30.48,66.68
  Bottom 0.3: IC2.22 34.98,62.98 33.78,64.18 33.78,64.73 33.43,65.08 30.79,65.08 R13.1
  Bottom 0.5: R13.1 R26.1
MASTER_RESET  (via drill 0.15 pad 0.3)  (1 unrouted)
  Top 1: S2.3 10.4,10.48 | 10.4,10.48 S2.1 | Q5.1 10.4,10.48
  Bottom 0.5: R37.1 11.95,10.7 Q5.1
  other vias: 12.18,10.48
N$1  (via drill 0.2 pad 0.4)  (1 unrouted)
  Bottom 0.3: v66.88,6.35 R28.1
N$2
  Bottom 0.3: Q2.3 62.98,6.35 R28.2
N$3
  Bottom 0.3: Q3.3 62.76,11.66 R29.2
N$4  (via drill 0.2 pad 0.4)  (1 unrouted)
  Bottom 0.3: v66.88,9.83 R29.1
N$5  (via drill 0.2 pad 0.4)  (1 unrouted)
  Bottom 0.3: v66.88,12.68 66.05,12.68 R30.1
N$6
  Bottom 0.3: J3.10 R34.1 R32.1
N$7
  Bottom 0.3: R33.1 10.69,19.59 J3.2
N$8  (via drill 0.15 pad 0.3)  (2 unrouted)
  Power/misc 0.5: v11.93,6.18 11.93,7.38 15.73,11.18 v17.33,11.18
  Bottom 0.5: D5.3 11.96,7.05 C20.1 | R100.1 17.13,11.43 Q4.2
N$9
  Bottom 0.5: R100.2 15.68,11.43 Q4.1 15.24,11.43 Q5.3
N$11
  Bottom 0.5: R38.1 16.81,3.49 Q6.1 14.5,4.54 C21.1
N$12
  Bottom 0.5: C22.1 R39.1 8.47,9.12 Q7.1
ON  (via drill 0.15 pad 0.3)  (3 unrouted)
  Top 0.3: R4.1 30.96,63.5 v30.93,63.53 | R27.2 6.34,102.87 C19.1
  Top 1: TP9.1 65.56,73.66 68.33,76.43 J4.3
  Power/fusetofuse1 0.3: v30.93,63.53 31.38,63.53 31.73,63.88 31.73,65.58 32.98,66.83 44.23,66.83 45.68,65.38 45.68,63.88 46.03,63.53 v46.33,63.53
  Power/fusetoio1 0.3: v30.93,63.53 31.08,63.53 31.48,63.93 31.48,82.86 14.02,100.33 9.42,100.33 7.42,102.33 v6.88,102.33
  Power/misc 0.3: v46.33,63.53 60.43,63.53 62.33,61.63 63.28,61.63 63.68,62.03 63.68,66.28 61.43,68.53 61.43,72.33 v62.78,73.68
  Bottom 0.3: R11.1 45.74,63.53 v46.33,63.53
  other vias: 72.58,76.43
ON1  (via drill 0.15 pad 0.3)  (1 unrouted)
  Top 0.3: IC1.4 34.73,62.48 33.71,63.5 R4.2 32.88,63.63 v32.38,63.63
  Power/fusetoio1 0.3: v14.48,55.23 23.43,55.23 28.48,60.28 28.48,61.83 29.58,62.93 31.73,62.93 32.38,63.58 v32.38,63.63
ON2  (via drill 0.15 pad 0.3)  (1 unrouted)
  Power/fusetoio2 0.3: v14.48,85.73 9.88,85.73 7.48,88.13 7.48,95.73 8.38,96.63 29.23,96.63 46.58,79.28 46.58,74.73 48.93,72.38 48.93,64.88 48.68,64.63 45.68,64.63 45.43,64.38 45.43,63.93 45.13,63.63 v44.88,63.63
  Bottom 0.3: IC2.4 42.58,62.48 43.6,63.5 R11.2 44.39,63.63 v44.88,63.63
ON_PRE_RES  (via drill 0.15 pad 0.3)  (1 unrouted)
  Bottom 1: v6.88,100.88 8.7,99.06 S1.2
SDA  (via drill 0.15 pad 0.3)  (3 unrouted)
  Top 0.2: IC1.6 35.18,61.48 34.73,61.03 v33.73,61.03
  Top 1: TP7.1 66.73,81.28 67.88,82.43 J4.1
  Power/fusetofuse1 0.3: v13.23,37.53 13.23,60.43 14.83,62.03 29.83,62.03 30.58,61.28 32.03,61.28 32.78,60.53 33.23,60.53 v33.73,61.03
  Power/misc 0.3: v33.73,61.03 33.73,59.43 35.23,57.93 42.13,57.93 43.58,59.38 v43.58,61.03 43.58,61.58 43.93,61.93 45.58,61.93 48.43,59.08 69.08,59.08 70.93,60.93 70.93,80.78 v72.53,82.38
  Bottom 0.2: IC2.6 42.18,61.48 42.63,61.03 v43.58,61.03
  other vias: 62.78,81.28
SLAVE_RESET  (via drill 0.15 pad 0.3)  (1 unrouted)
  Top 1: J4.6 71.13,67.43 65.93,62.23 TP12.1 59.53,62.23 56.58,59.28 56.58,51.63 72.98,35.23 72.98,7.72 66.3,1.03 20.48,1.03 v14.48,7.03
  Bottom 0.5: C22.2 12.66,8.89 C21.2 14.57,6.98 R36.1 15.68,8.38 Q4.3
SS  (via drill 0.15 pad 0.3)  (4 unrouted)
  Top 1: TP13.1 70.37,58.42 70.49,58.3 J5.1
  Power/fusetofuse1 0.3: v45.83,60.58 45.83,59.69 | 45.83,59.69 45.83,59.63 | v31.43,60.58 31.43,59.68 32.38,58.74 32.92,58.74 33.63,58.03 43.32,58.03 43.71,58.42 44.56,58.42 45.83,59.69
  Power/misc 0.3: v45.83,60.58 47.98,58.43 v62.73,58.43
  other vias: 72.53,58.28
SS1  (via drill 0.15 pad 0.3)  (2 unrouted)
  Top 0.3: IC1.19 44.17,61.48 44.25,61.56 C14.1
  Top 0.5: R8.1 44.26,61.55 44.25,61.56
  Power/fusetoio1 0.3: v9.43,49.48 7.28,47.33 7.28,41.63 8.53,40.38 23.73,40.38 29.43,46.08 29.43,50.38 29.88,50.83 36.08,50.83 37.38,52.13 44.08,52.13 44.88,52.93 44.88,58.23 44.28,58.83 v44.28,61.28
SS2  (via drill 0.15 pad 0.3)  (2 unrouted)
  Power/fusetoio2 0.3: v9.43,80.03 28.28,80.03 28.78,79.53 28.78,72.13 26.98,70.33 26.98,65.58 29.58,62.98 31.78,62.98 32.98,61.78 v32.98,61.28
  Bottom 0.3: IC2.19 33.1,61.48 C17.1
  Bottom 0.5: R15.1 33.01,61.39 33.1,61.48
TP29
  Top 0.3: TP1.1 15.77,33.02 J3.7
TP30
  Top 0.3: TP2.1 11.96,29.21 J3.8
VDD1  (via drill 0.15 pad 0.3)  (3 unrouted)
  Top 0.3: IC1.21 42.78,62.48 43.17,62.86 C13.1 44.28,63.78 44.63,64.13 v44.93,64.13
  Power/fusetoio1 0.3: v9.43,53.33 6.58,50.48 6.58,41.38 8.13,39.83 24.43,39.83 31.73,47.13 45.63,47.13 46.38,47.88 46.38,52.13 47.13,52.88 48.58,52.88 48.98,53.28 48.98,56.68 45.03,60.63 45.03,62.48 44.33,63.18 44.33,63.82 44.65,64.13 v44.93,64.13
  Power/misc 0.5: v13.43,2.53 10.38,2.53 4.73,8.18 4.73,48.63 v9.43,53.33
  Bottom 0.5: D5.2 D5.1 13.45,3.44 Q6.3
VDD2  (via drill 0.15 pad 0.3)  (3 unrouted)
  Power/fusetoio2 0.3: v9.43,83.83 28.38,83.83 29.53,82.68 29.53,71.63 28.18,70.28 28.18,66.93 29.73,65.38 31.23,65.38 31.68,64.93 31.68,64.33 31.88,64.13 v32.33,64.13
  Power/misc 0.5: v7.53,12.48 7.53,49.63 10.63,52.73 10.63,82.63 v9.43,83.83
  Bottom 0.3: IC2.21 34.63,62.48 34.25,62.86 C16.1 32.98,63.93 32.79,64.13 v32.33,64.13
  Bottom 0.5: C16.1 33.01,62.89
VIN  (via drill 0.15 pad 0.3)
